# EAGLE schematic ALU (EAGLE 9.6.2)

## Sheet 1 of 8: Motherboard
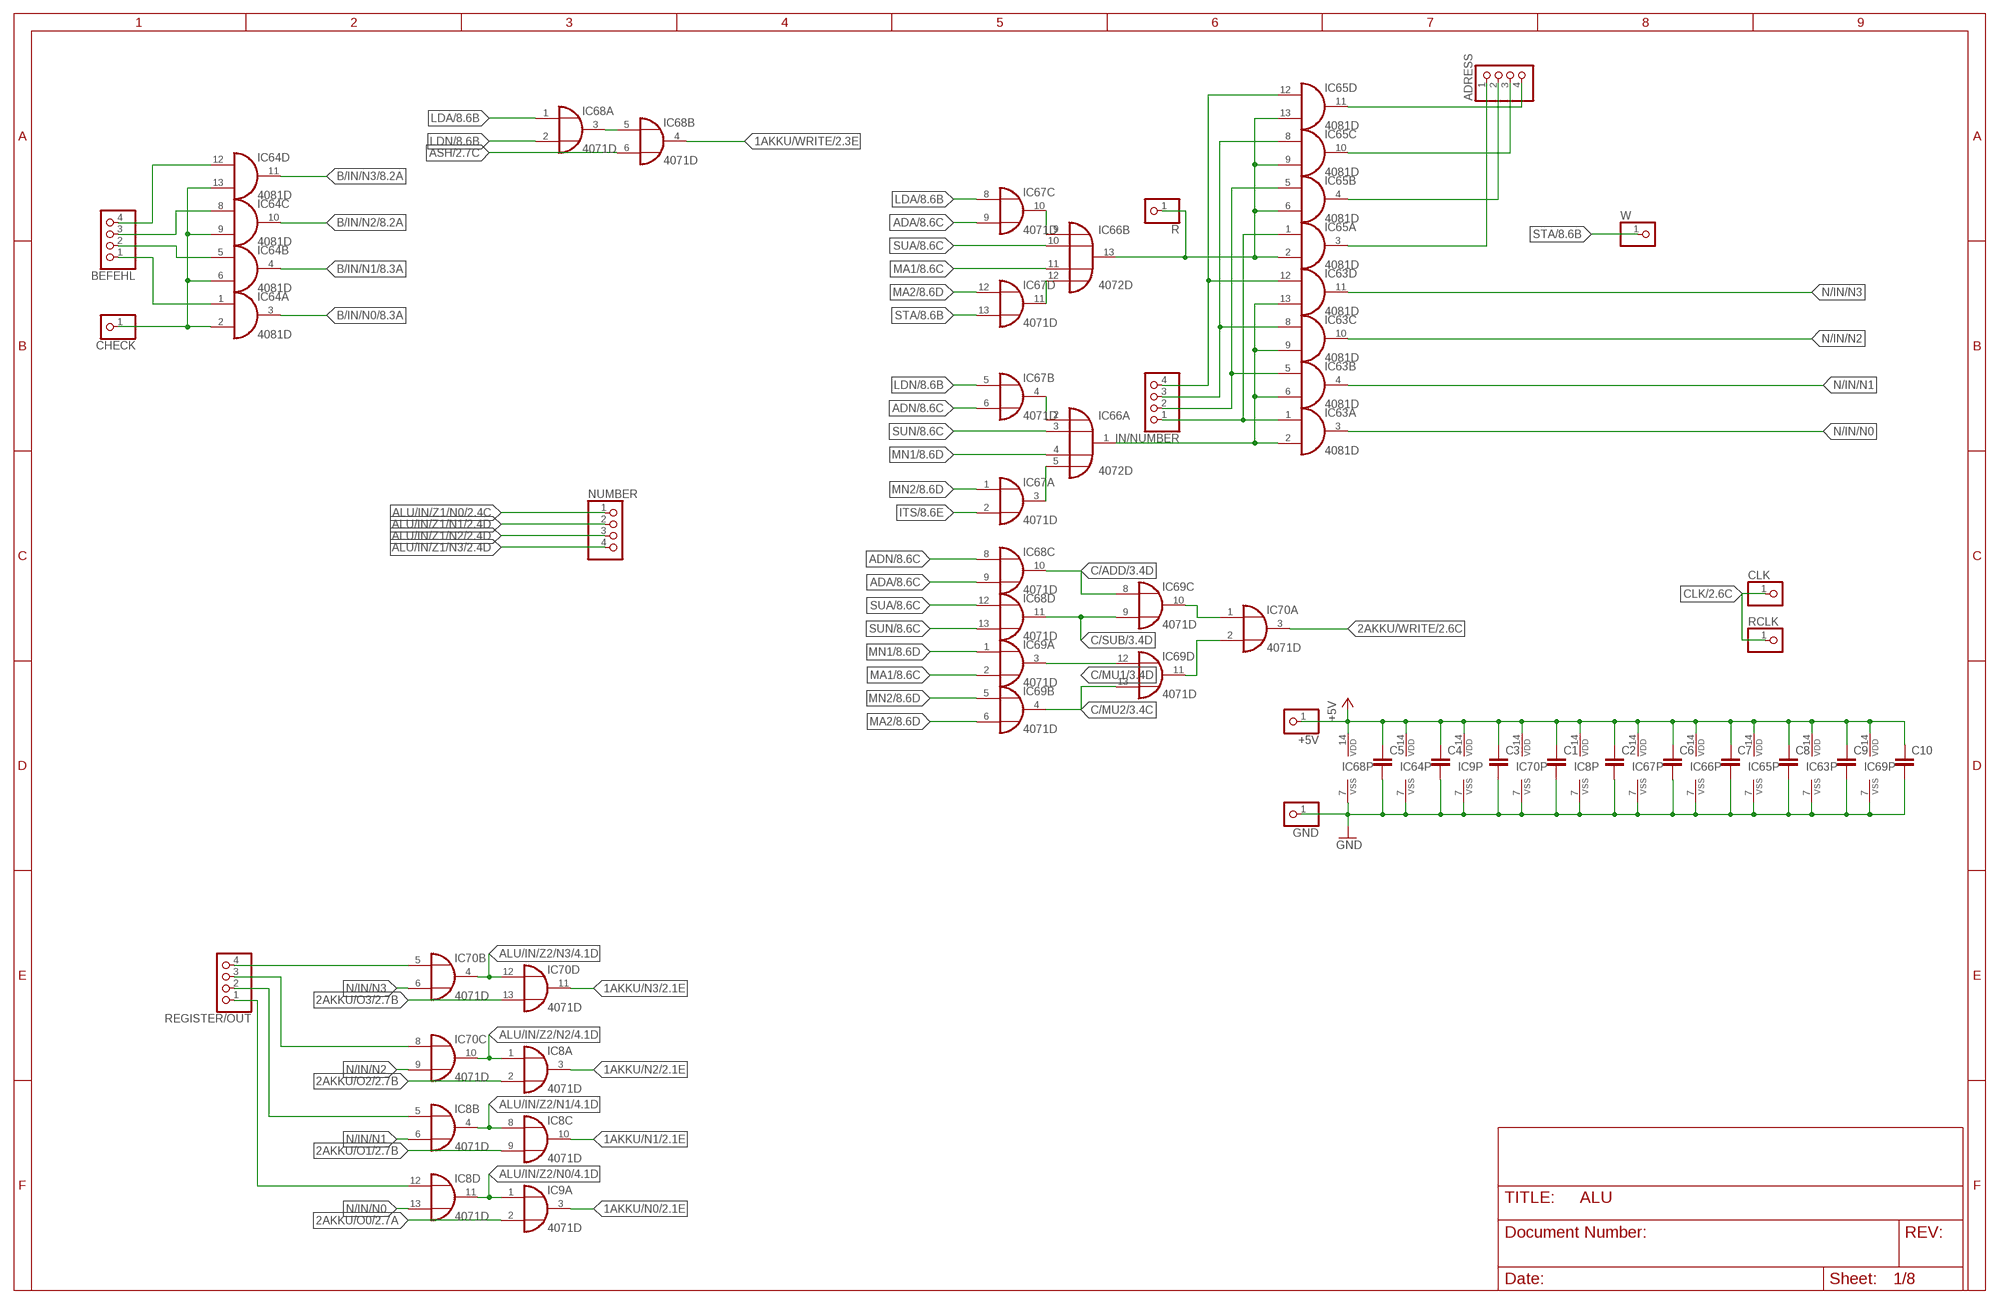
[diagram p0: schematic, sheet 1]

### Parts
+5V  PINHD-1X1  [1X01]
ADRESS  PINHD-1X4  [1X04]
BEFEHL  PINHD-1X4  [1X04]
C1  C-EUC0805  [C0805]
C2  C-EUC0805  [C0805]
C3  C-EUC0805  [C0805]
C4  C-EUC0805  [C0805]
C5  C-EUC0805  [C0805]
C6  C-EUC0805  [C0805]
C7  C-EUC0805  [C0805]
C8  C-EUC0805  [C0805]
C9  C-EUC0805  [C0805]
C10  C-EUC0805  [C0805]
CHECK  PINHD-1X1  [1X01]
CLK  PINHD-1X1  [1X01]
GND  PINHD-1X1  [1X01]
IC8  4071D  [SO14]
IC9  4071D  [SO14]
IC63  4081D  [SO14]
IC64  4081D  [SO14]
IC65  4081D  [SO14]
IC66  4072D  [SO14]
IC67  4071D  [SO14]
IC68  4071D  [SO14]
IC69  4071D  [SO14]
IC70  4071D  [SO14]
IN/NUMBER  PINHD-1X4  [1X04]
NUMBER  PINHD-1X4  [1X04]
R  PINHD-1X1  [1X01]
RCLK  PINHD-1X1  [1X01]
REGISTER/OUT  PINHD-1X4  [1X04]
W  PINHD-1X1  [1X01]

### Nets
1AKKU/N0: IC9.3(A:O) ; also sheet 2
1AKKU/N1: IC8.10(C:O) ; also sheet 2
1AKKU/N2: IC8.3(A:O) ; also sheet 2
1AKKU/N3: IC70.11(D:O) ; also sheet 2
1AKKU/WRITE: IC68.4(B:O) ; also sheet 2
2AKKU/O0: IC9.2(A:I1) ; also sheet 2
2AKKU/O1: IC8.9(C:I1) ; also sheet 2
2AKKU/O2: IC8.2(A:I1) ; also sheet 2
2AKKU/O3: IC70.13(D:I1) ; also sheet 2
2AKKU/WRITE: IC70.3(A:O) ; also sheet 2
+5V: +5V.1 C1.1 C2.1 C3.1 C4.1 C5.1 C6.1 C7.1 C8.1 C9.1 C10.1 IC8.14(P:VDD) IC9.14(P:VDD) IC63.14(P:VDD) IC64.14(P:VDD) IC65.14(P:VDD) IC66.14(P:VDD) IC67.14(P:VDD) IC68.14(P:VDD) IC69.14(P:VDD) IC70.14(P:VDD) ; also sheet 2,3,4,5,6,7,8
A/IN/N0: ADRESS.1 IC65.3(A:O)
A/IN/N1: ADRESS.2 IC65.4(B:O)
A/IN/N2: ADRESS.3 IC65.10(C:O)
A/IN/N3: ADRESS.4 IC65.11(D:O)
ADA: IC67.9(C:I1) IC68.9(C:I1) ; also sheet 8
ADN: IC67.6(B:I1) IC68.8(C:I0) ; also sheet 8
ALU/IN/Z1/N0: NUMBER.1 ; also sheet 2,4,5,6,7
ALU/IN/Z1/N1: NUMBER.2 ; also sheet 2,4,5,6,7
ALU/IN/Z1/N2: NUMBER.3 ; also sheet 2,4,5,6,7
ALU/IN/Z1/N3: NUMBER.4 ; also sheet 2,4,5,6,7
ALU/IN/Z2/N0: IC8.11(D:O) IC9.1(A:I0) ; also sheet 4,5,6,7
ALU/IN/Z2/N1: IC8.4(B:O) IC8.8(C:I0) ; also sheet 4,5,6,7
ALU/IN/Z2/N2: IC8.1(A:I0) IC70.10(C:O) ; also sheet 4,5,6,7
ALU/IN/Z2/N3: IC70.4(B:O) IC70.12(D:I0) ; also sheet 4,5,6,7
ASH: IC68.6(B:I1) ; also sheet 2,8
B/IN/N0: IC64.3(A:O) ; also sheet 8
B/IN/N1: IC64.4(B:O) ; also sheet 8
B/IN/N2: IC64.10(C:O) ; also sheet 8
B/IN/N3: IC64.11(D:O) ; also sheet 8
C/ADD: IC68.10(C:O) IC69.8(C:I0) ; also sheet 3
C/MU1: IC69.3(A:O) IC69.12(D:I0) ; also sheet 3
C/MU2: IC69.4(B:O) IC69.13(D:I1) ; also sheet 3
C/SUB: IC68.11(D:O) IC69.9(C:I1) ; also sheet 3
CLK: CLK.1 RCLK.1 ; also sheet 2,3
GND: C1.2 C2.2 C3.2 C4.2 C5.2 C6.2 C7.2 C8.2 C9.2 C10.2 GND.1 IC8.7(P:VSS) IC9.7(P:VSS) IC63.7(P:VSS) IC64.7(P:VSS) IC65.7(P:VSS) IC66.7(P:VSS) IC67.7(P:VSS) IC68.7(P:VSS) IC69.7(P:VSS) IC70.7(P:VSS) ; also sheet 2,3,4,5,6,7,8
ITS: IC67.2(A:I1) ; also sheet 8
LDA: IC67.8(C:I0) IC68.1(A:I0) ; also sheet 8
LDN: IC67.5(B:I0) IC68.2(A:I1) ; also sheet 8
MA1: IC66.11(B:I2) IC69.2(A:I1) ; also sheet 8
MA2: IC67.12(D:I0) IC69.6(B:I1) ; also sheet 8
MN1: IC66.4(A:I2) IC69.1(A:I0) ; also sheet 8
MN2: IC67.1(A:I0) IC69.5(B:I0) ; also sheet 8
N$14: IC70.5(B:I0) REGISTER/OUT.4
N$19: IC70.8(C:I0) REGISTER/OUT.3
N$20: IC8.5(B:I0) REGISTER/OUT.2
N$22: IC8.12(D:I0) REGISTER/OUT.1
N$141: BEFEHL.4 IC64.12(D:I0)
N$143: BEFEHL.3 IC64.8(C:I0)
N$145: BEFEHL.2 IC64.5(B:I0)
N$147: BEFEHL.1 IC64.1(A:I0)
N$149: CHECK.1 IC64.2(A:I1) IC64.6(B:I1) IC64.9(C:I1) IC64.13(D:I1)
N$150: IC63.12(D:I0) IC65.12(D:I0) IN/NUMBER.4
N$151: IC63.8(C:I0) IC65.8(C:I0) IN/NUMBER.3
N$152: IC63.5(B:I0) IC65.5(B:I0) IN/NUMBER.2
N$153: IC63.1(A:I0) IC65.1(A:I0) IN/NUMBER.1
N$154: IC63.2(A:I1) IC63.6(B:I1) IC63.9(C:I1) IC63.13(D:I1) IC66.1(A:O)
N$155: IC68.3(A:O) IC68.5(B:I0)
N$156: IC66.5(A:I3) IC67.3(A:O)
N$158: IC66.2(A:I0) IC67.4(B:O)
N$159: IC65.2(A:I1) IC65.6(B:I1) IC65.9(C:I1) IC65.13(D:I1) IC66.13(B:O) R.1
N$160: IC66.9(B:I0) IC67.10(C:O)
N$161: IC66.12(B:I3) IC67.11(D:O)
N$173: IC69.10(C:O) IC70.1(A:I0)
N$174: IC69.11(D:O) IC70.2(A:I1)
N/IN/N0: IC8.13(D:I1) IC63.3(A:O)
N/IN/N1: IC8.6(B:I1) IC63.4(B:O)
N/IN/N2: IC63.10(C:O) IC70.9(C:I1)
N/IN/N3: IC63.11(D:O) IC70.6(B:I1)
STA: IC67.13(D:I1) W.1 ; also sheet 8
SUA: IC66.10(B:I1) IC68.12(D:I0) ; also sheet 8
SUN: IC66.3(A:I1) IC68.13(D:I1) ; also sheet 8

## Sheet 2 of 8: Akkumulator
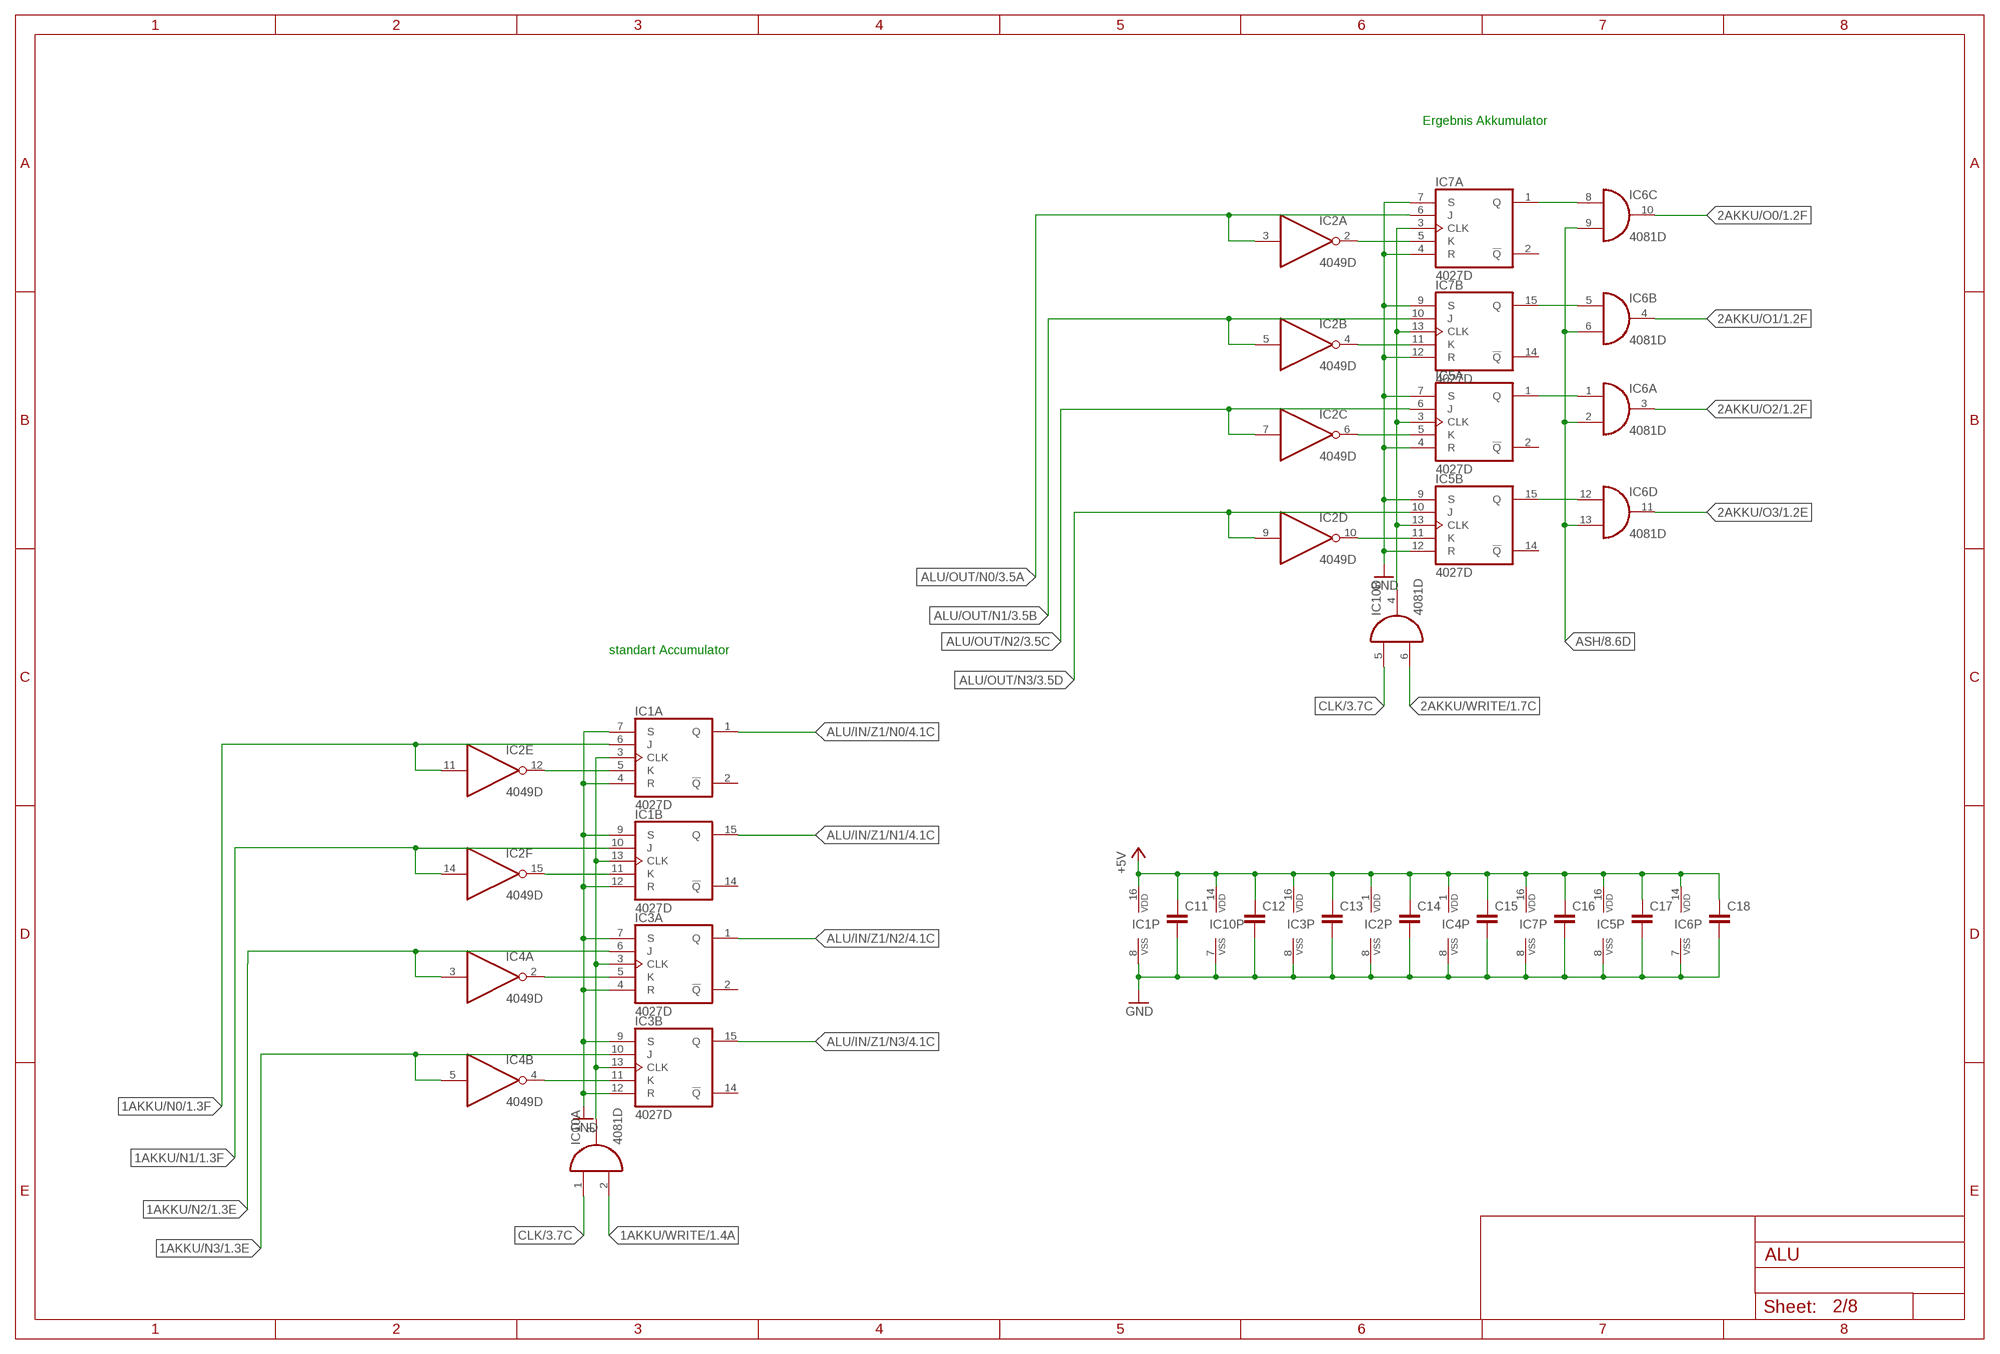
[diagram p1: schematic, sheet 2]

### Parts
C11  C-EUC0805  [C0805]
C12  C-EUC0805  [C0805]
C13  C-EUC0805  [C0805]
C14  C-EUC0805  [C0805]
C15  C-EUC0805  [C0805]
C16  C-EUC0805  [C0805]
C17  C-EUC0805  [C0805]
C18  C-EUC0805  [C0805]
IC1  4027D  [SO16]
IC2  4049D  [SO16]
IC3  4027D  [SO16]
IC4  4049D  [SO16]
IC5  4027D  [SO16]
IC6  4081D  [SO14]
IC7  4027D  [SO16]
IC10  4081D  [SO14]

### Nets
1AKKU/N0: IC1.6(A:J) IC2.11(E:I) ; also sheet 1
1AKKU/N1: IC1.10(B:J) IC2.14(F:I) ; also sheet 1
1AKKU/N2: IC3.6(A:J) IC4.3(A:I) ; also sheet 1
1AKKU/N3: IC3.10(B:J) IC4.5(B:I) ; also sheet 1
1AKKU/WRITE: IC10.2(A:I1) ; also sheet 1
2AKKU/O0: IC6.10(C:O) ; also sheet 1
2AKKU/O1: IC6.4(B:O) ; also sheet 1
2AKKU/O2: IC6.3(A:O) ; also sheet 1
2AKKU/O3: IC6.11(D:O) ; also sheet 1
2AKKU/WRITE: IC10.6(B:I1) ; also sheet 1
+5V: C11.1 C12.1 C13.1 C14.1 C15.1 C16.1 C17.1 C18.1 IC1.16(P:VDD) IC2.1(P:VDD) IC3.16(P:VDD) IC4.1(P:VDD) IC5.16(P:VDD) IC6.14(P:VDD) IC7.16(P:VDD) IC10.14(P:VDD) ; also sheet 1,3,4,5,6,7,8
ALU/IN/Z1/N0: IC1.1(A:Q) ; also sheet 1,4,5,6,7
ALU/IN/Z1/N1: IC1.15(B:Q) ; also sheet 1,4,5,6,7
ALU/IN/Z1/N2: IC3.1(A:Q) ; also sheet 1,4,5,6,7
ALU/IN/Z1/N3: IC3.15(B:Q) ; also sheet 1,4,5,6,7
ALU/OUT/N0: IC2.3(A:I) IC7.6(A:J) ; also sheet 3
ALU/OUT/N1: IC2.5(B:I) IC7.10(B:J) ; also sheet 3
ALU/OUT/N2: IC2.7(C:I) IC5.6(A:J) ; also sheet 3
ALU/OUT/N3: IC2.9(D:I) IC5.10(B:J) ; also sheet 3
ASH: IC6.2(A:I1) IC6.6(B:I1) IC6.9(C:I1) IC6.13(D:I1) ; also sheet 1,8
CLK: IC10.1(A:I0) IC10.5(B:I0) ; also sheet 1,3
GND: C11.2 C12.2 C13.2 C14.2 C15.2 C16.2 C17.2 C18.2 IC1.4(A:R) IC1.7(A:S) IC1.8(P:VSS) IC1.9(B:S) IC1.12(B:R) IC2.8(P:VSS) IC3.4(A:R) IC3.7(A:S) IC3.8(P:VSS) IC3.9(B:S) IC3.12(B:R) IC4.8(P:VSS) IC5.4(A:R) IC5.7(A:S) IC5.8(P:VSS) IC5.9(B:S) IC5.12(B:R) IC6.7(P:VSS) IC7.4(A:R) IC7.7(A:S) IC7.8(P:VSS) IC7.9(B:S) IC7.12(B:R) IC10.7(P:VSS) ; also sheet 1,3,4,5,6,7,8
N$1: IC1.5(A:K) IC2.12(E:O)
N$2: IC5.3(A:CLK) IC5.13(B:CLK) IC7.3(A:CLK) IC7.13(B:CLK) IC10.4(B:O)
N$3: IC1.3(A:CLK) IC1.13(B:CLK) IC3.3(A:CLK) IC3.13(B:CLK) IC10.3(A:O)
N$4: IC1.11(B:K) IC2.15(F:O)
N$5: IC3.5(A:K) IC4.2(A:O)
N$6: IC6.8(C:I0) IC7.1(A:Q)
N$7: IC6.5(B:I0) IC7.15(B:Q)
N$8: IC3.11(B:K) IC4.4(B:O)
N$9: IC2.6(C:O) IC5.5(A:K)
N$10: IC5.1(A:Q) IC6.1(A:I0)
N$11: IC5.15(B:Q) IC6.12(D:I0)
N$12: IC2.10(D:O) IC5.11(B:K)
N$13: IC2.2(A:O) IC7.5(A:K)
N$16: IC2.4(B:O) IC7.11(B:K)
Unconnected: IC1.2(A:!Q) IC1.14(B:!Q) IC3.2(A:!Q) IC3.14(B:!Q) IC5.2(A:!Q) IC5.14(B:!Q) IC7.2(A:!Q) IC7.14(B:!Q)

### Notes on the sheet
- Ergebnis Akkumulator
- standart Accumulator

## Sheet 3 of 8: ALU
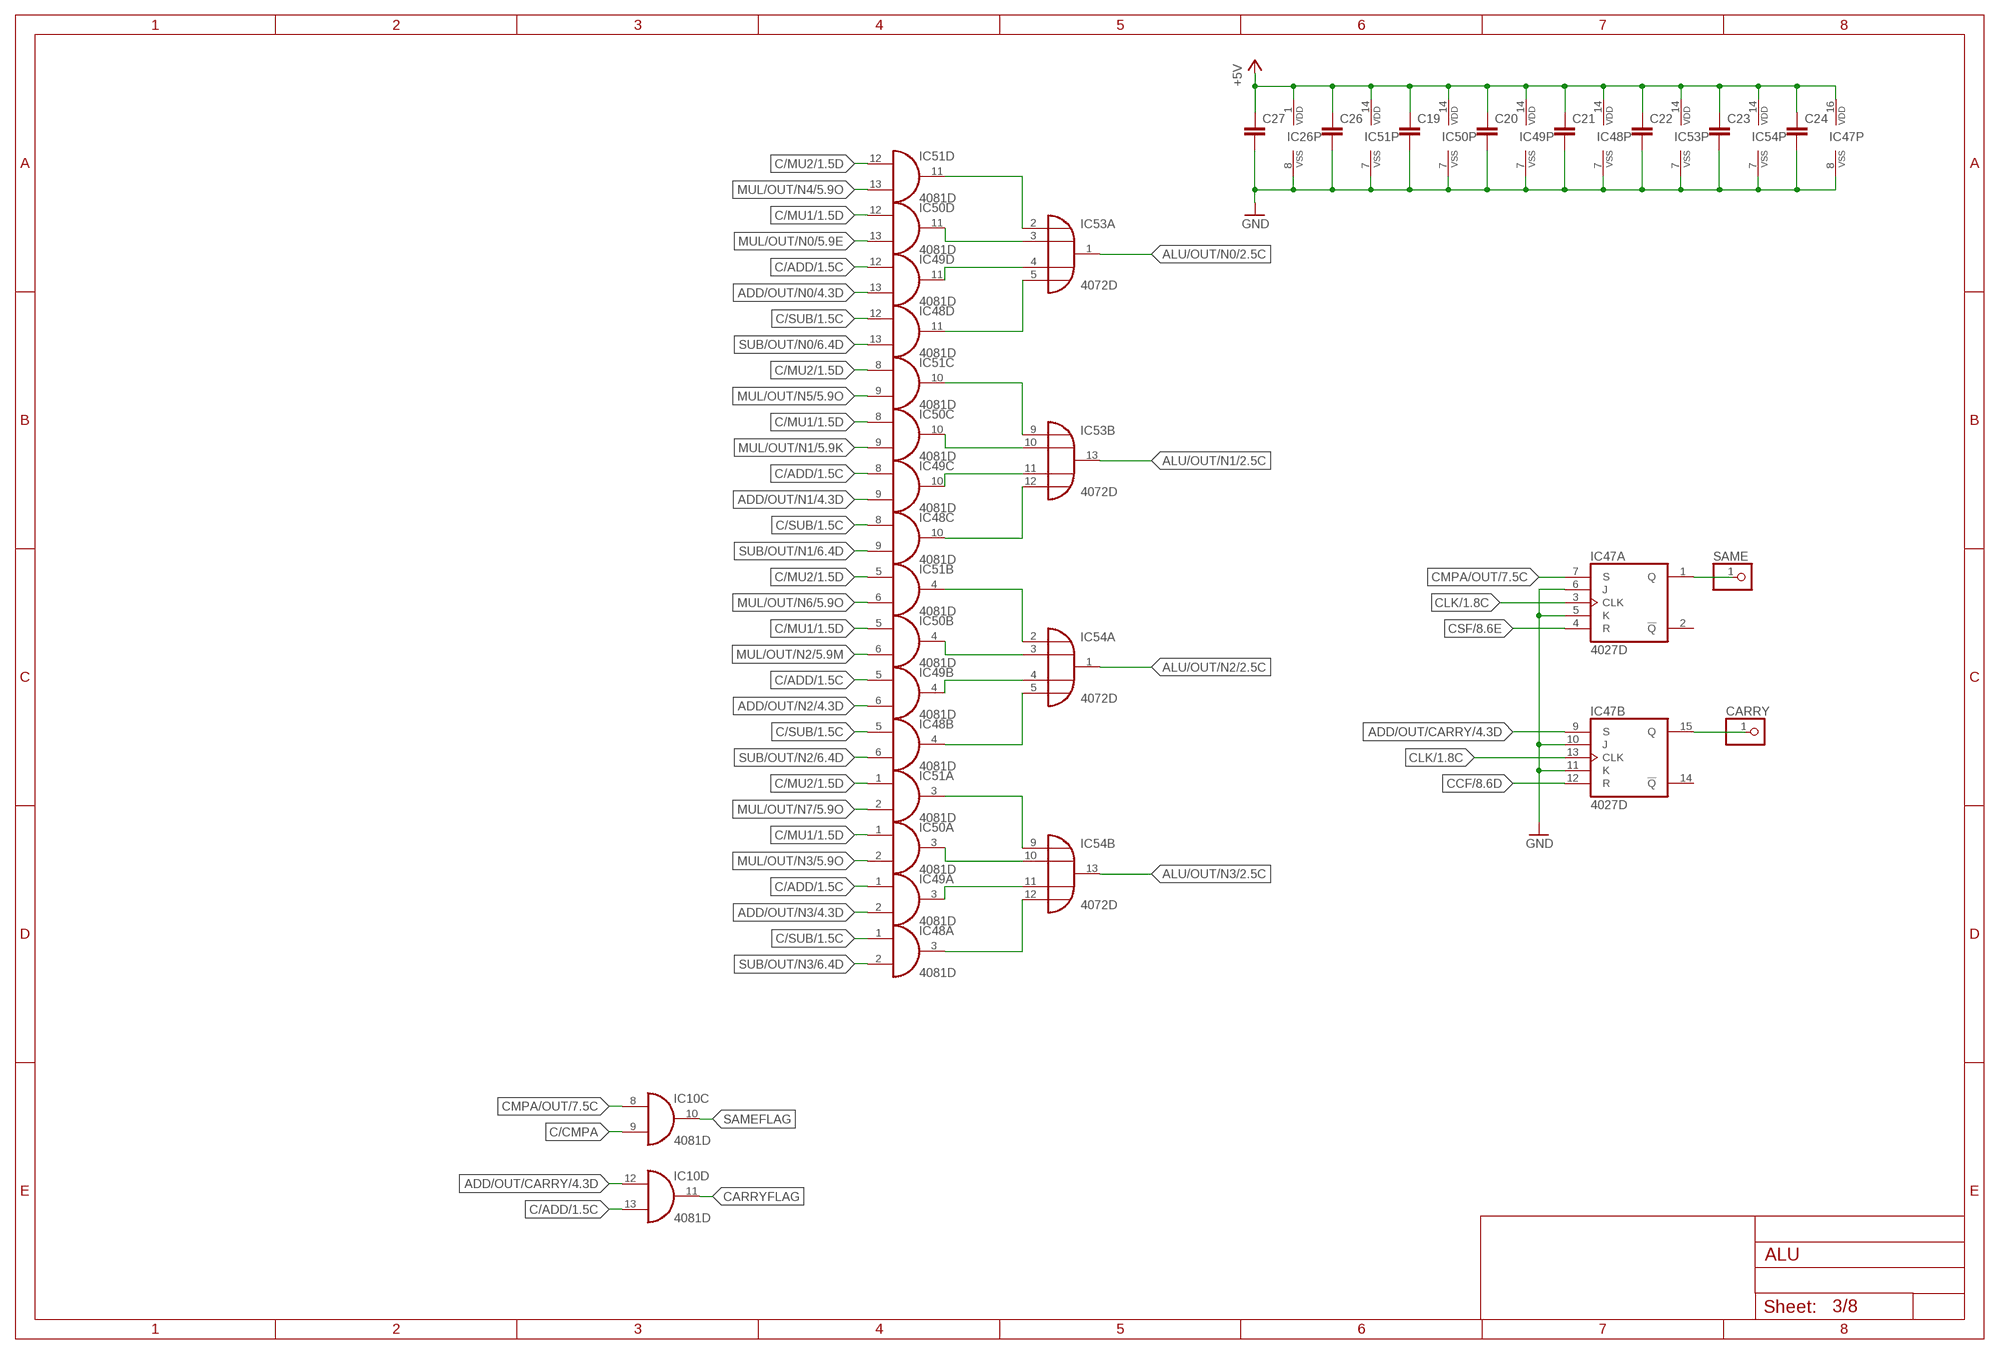
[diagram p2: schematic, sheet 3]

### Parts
C19  C-EUC0805  [C0805]
C20  C-EUC0805  [C0805]
C21  C-EUC0805  [C0805]
C22  C-EUC0805  [C0805]
C23  C-EUC0805  [C0805]
C24  C-EUC0805  [C0805]
C26  C-EUC0805  [C0805]
C27  C-EUC0805  [C0805]
CARRY  PINHD-1X1  [1X01]
IC26  4049D  [SO16]
IC47  4027D  [SO16]
IC48  4081D  [SO14]
IC49  4081D  [SO14]
IC50  4081D  [SO14]
IC51  4081D  [SO14]
IC53  4072D  [SO14]
IC54  4072D  [SO14]
SAME  PINHD-1X1  [1X01]

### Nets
+5V: C19.1 C20.1 C21.1 C22.1 C23.1 C24.1 C26.1 C27.1 IC26.1(P:VDD) IC47.16(P:VDD) IC48.14(P:VDD) IC49.14(P:VDD) IC50.14(P:VDD) IC51.14(P:VDD) IC53.14(P:VDD) IC54.14(P:VDD) ; also sheet 1,2,4,5,6,7,8
ADD/OUT/CARRY: IC10.12(D:I0) IC47.9(B:S) ; also sheet 4
ADD/OUT/N0: IC49.13(D:I1) ; also sheet 4
ADD/OUT/N1: IC49.9(C:I1) ; also sheet 4
ADD/OUT/N2: IC49.6(B:I1) ; also sheet 4
ADD/OUT/N3: IC49.2(A:I1) ; also sheet 4
ALU/OUT/N0: IC53.1(A:O) ; also sheet 2
ALU/OUT/N1: IC53.13(B:O) ; also sheet 2
ALU/OUT/N2: IC54.1(A:O) ; also sheet 2
ALU/OUT/N3: IC54.13(B:O) ; also sheet 2
C/ADD: IC10.13(D:I1) IC49.1(A:I0) IC49.5(B:I0) IC49.8(C:I0) IC49.12(D:I0) ; also sheet 1
C/CMPA: IC10.9(C:I1)
C/MU1: IC50.1(A:I0) IC50.5(B:I0) IC50.8(C:I0) IC50.12(D:I0) ; also sheet 1
C/MU2: IC51.1(A:I0) IC51.5(B:I0) IC51.8(C:I0) IC51.12(D:I0) ; also sheet 1
C/SUB: IC48.1(A:I0) IC48.5(B:I0) IC48.8(C:I0) IC48.12(D:I0) ; also sheet 1
CARRYFLAG: IC10.11(D:O)
CCF: IC47.12(B:R) ; also sheet 8
CLK: IC47.3(A:CLK) IC47.13(B:CLK) ; also sheet 1,2
CMPA/OUT: IC10.8(C:I0) IC47.7(A:S) ; also sheet 7
CSF: IC47.4(A:R) ; also sheet 8
GND: C19.2 C20.2 C21.2 C22.2 C23.2 C24.2 C26.2 C27.2 IC26.8(P:VSS) IC47.5(A:K) IC47.6(A:J) IC47.8(P:VSS) IC47.10(B:J) IC47.11(B:K) IC48.7(P:VSS) IC49.7(P:VSS) IC50.7(P:VSS) IC51.7(P:VSS) IC53.7(P:VSS) IC54.7(P:VSS) ; also sheet 1,2,4,5,6,7,8
MUL/OUT/N0: IC50.13(D:I1) ; also sheet 5
MUL/OUT/N1: IC50.9(C:I1) ; also sheet 5
MUL/OUT/N2: IC50.6(B:I1) ; also sheet 5
MUL/OUT/N3: IC50.2(A:I1) ; also sheet 5
MUL/OUT/N4: IC51.13(D:I1) ; also sheet 5
MUL/OUT/N5: IC51.9(C:I1) ; also sheet 5
MUL/OUT/N6: IC51.6(B:I1) ; also sheet 5
MUL/OUT/N7: IC51.2(A:I1) ; also sheet 5
N$106: IC49.11(D:O) IC53.4(A:I2)
N$120: IC50.11(D:O) IC53.3(A:I1)
N$121: IC51.11(D:O) IC53.2(A:I0)
N$122: IC48.11(D:O) IC53.5(A:I3)
N$123: IC49.10(C:O) IC53.11(B:I2)
N$124: IC50.10(C:O) IC53.10(B:I1)
N$125: IC51.10(C:O) IC53.9(B:I0)
N$126: IC48.10(C:O) IC53.12(B:I3)
N$133: IC50.4(B:O) IC54.3(A:I1)
N$134: IC49.4(B:O) IC54.4(A:I2)
N$135: IC48.4(B:O) IC54.5(A:I3)
N$136: IC51.4(B:O) IC54.2(A:I0)
N$137: IC50.3(A:O) IC54.10(B:I1)
N$138: IC49.3(A:O) IC54.11(B:I2)
N$139: IC51.3(A:O) IC54.9(B:I0)
N$140: IC48.3(A:O) IC54.12(B:I3)
N$167: IC47.1(A:Q) SAME.1
N$171: CARRY.1 IC47.15(B:Q)
SAMEFLAG: IC10.10(C:O)
SUB/OUT/N0: IC48.13(D:I1) ; also sheet 6
SUB/OUT/N1: IC48.9(C:I1) ; also sheet 6
SUB/OUT/N2: IC48.6(B:I1) ; also sheet 6
SUB/OUT/N3: IC48.2(A:I1) ; also sheet 6
Unconnected: IC47.2(A:!Q) IC47.14(B:!Q)

## Sheet 4 of 8: Addirer
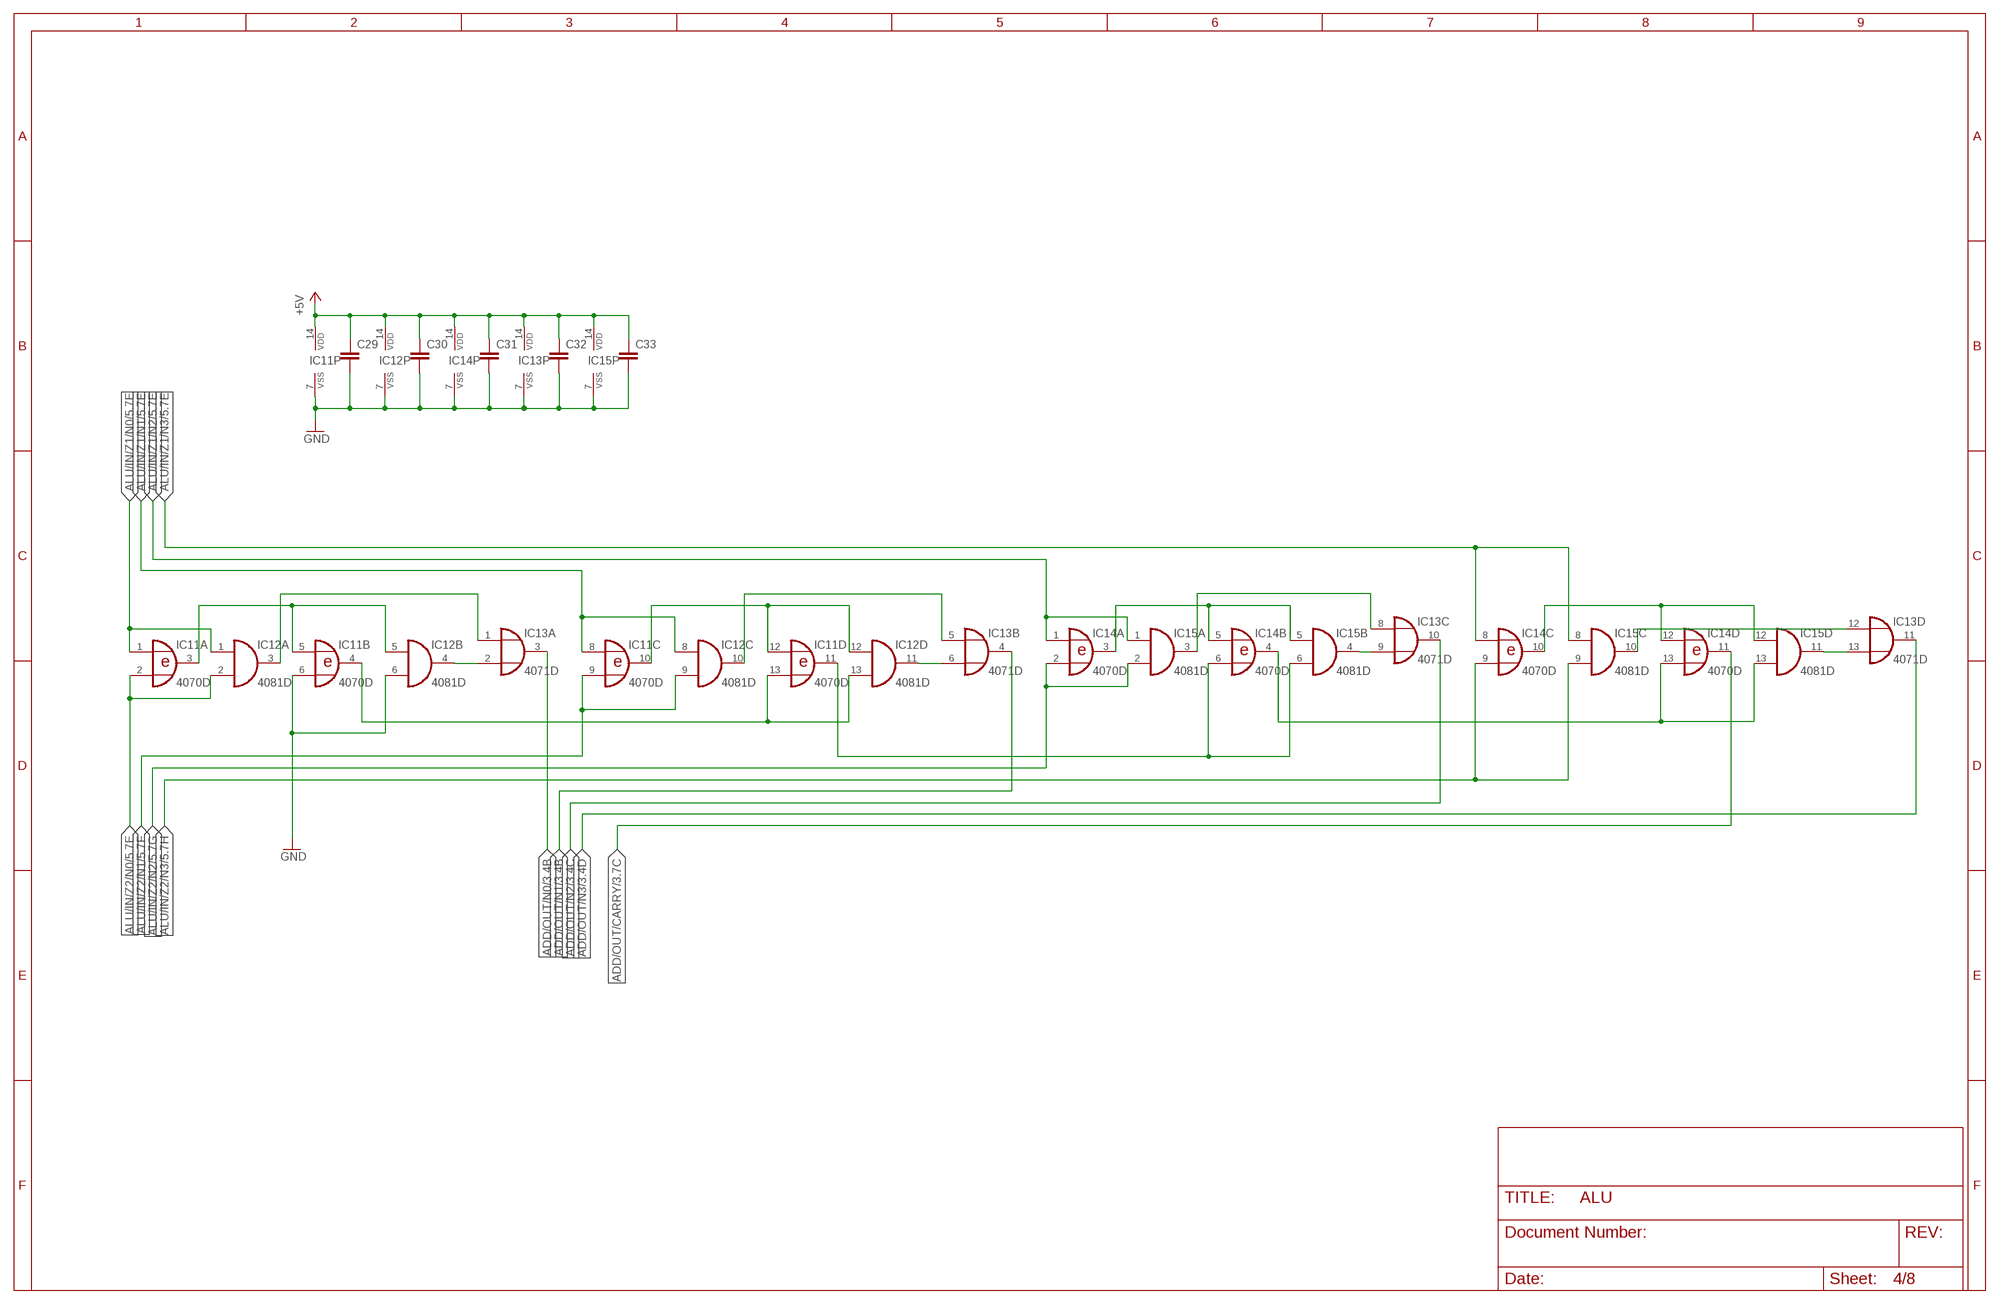
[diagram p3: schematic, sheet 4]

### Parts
C29  C-EUC0805  [C0805]
C30  C-EUC0805  [C0805]
C31  C-EUC0805  [C0805]
C32  C-EUC0805  [C0805]
C33  C-EUC0805  [C0805]
IC11  4070D  [SO14]
IC12  4081D  [SO14]
IC13  4071D  [SO14]
IC14  4070D  [SO14]
IC15  4081D  [SO14]

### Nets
+5V: C29.1 C30.1 C31.1 C32.1 C33.1 IC11.14(P:VDD) IC12.14(P:VDD) IC13.14(P:VDD) IC14.14(P:VDD) IC15.14(P:VDD) ; also sheet 1,2,3,5,6,7,8
ADD/OUT/CARRY: IC14.11(D:O) ; also sheet 3
ADD/OUT/N0: IC13.3(A:O) ; also sheet 3
ADD/OUT/N1: IC13.4(B:O) ; also sheet 3
ADD/OUT/N2: IC13.10(C:O) ; also sheet 3
ADD/OUT/N3: IC13.11(D:O) ; also sheet 3
ALU/IN/Z1/N0: IC11.1(A:I0) IC12.1(A:I0) ; also sheet 1,2,5,6,7
ALU/IN/Z1/N1: IC11.8(C:I0) IC12.8(C:I0) ; also sheet 1,2,5,6,7
ALU/IN/Z1/N2: IC14.1(A:I0) IC15.1(A:I0) ; also sheet 1,2,5,6,7
ALU/IN/Z1/N3: IC14.8(C:I0) IC15.8(C:I0) ; also sheet 1,2,5,6,7
ALU/IN/Z2/N0: IC11.2(A:I1) IC12.2(A:I1) ; also sheet 1,5,6,7
ALU/IN/Z2/N1: IC11.9(C:I1) IC12.9(C:I1) ; also sheet 1,5,6,7
ALU/IN/Z2/N2: IC14.2(A:I1) IC15.2(A:I1) ; also sheet 1,5,6,7
ALU/IN/Z2/N3: IC14.9(C:I1) IC15.9(C:I1) ; also sheet 1,5,6,7
GND: C29.2 C30.2 C31.2 C32.2 C33.2 IC11.6(B:I1) IC11.7(P:VSS) IC12.6(B:I1) IC12.7(P:VSS) IC13.7(P:VSS) IC14.7(P:VSS) IC15.7(P:VSS) ; also sheet 1,2,3,5,6,7,8
N$21: IC11.3(A:O) IC11.5(B:I0) IC12.5(B:I0)
N$25: IC12.3(A:O) IC13.1(A:I0)
N$29: IC12.4(B:O) IC13.2(A:I1)
N$31: IC11.4(B:O) IC11.13(D:I1) IC12.13(D:I1)
N$39: IC11.11(D:O) IC14.6(B:I1) IC15.6(B:I1)
N$40: IC11.10(C:O) IC11.12(D:I0) IC12.12(D:I0)
N$41: IC12.10(C:O) IC13.5(B:I0)
N$42: IC12.11(D:O) IC13.6(B:I1)
N$48: IC14.3(A:O) IC14.5(B:I0) IC15.5(B:I0)
N$49: IC14.4(B:O) IC14.13(D:I1) IC15.13(D:I1)
N$50: IC13.9(C:I1) IC15.4(B:O)
N$51: IC13.8(C:I0) IC15.3(A:O)
N$54: IC14.10(C:O) IC14.12(D:I0) IC15.12(D:I0)
N$55: IC13.12(D:I0) IC15.10(C:O)
N$56: IC13.13(D:I1) IC15.11(D:O)

## Sheet 5 of 8: multiplier
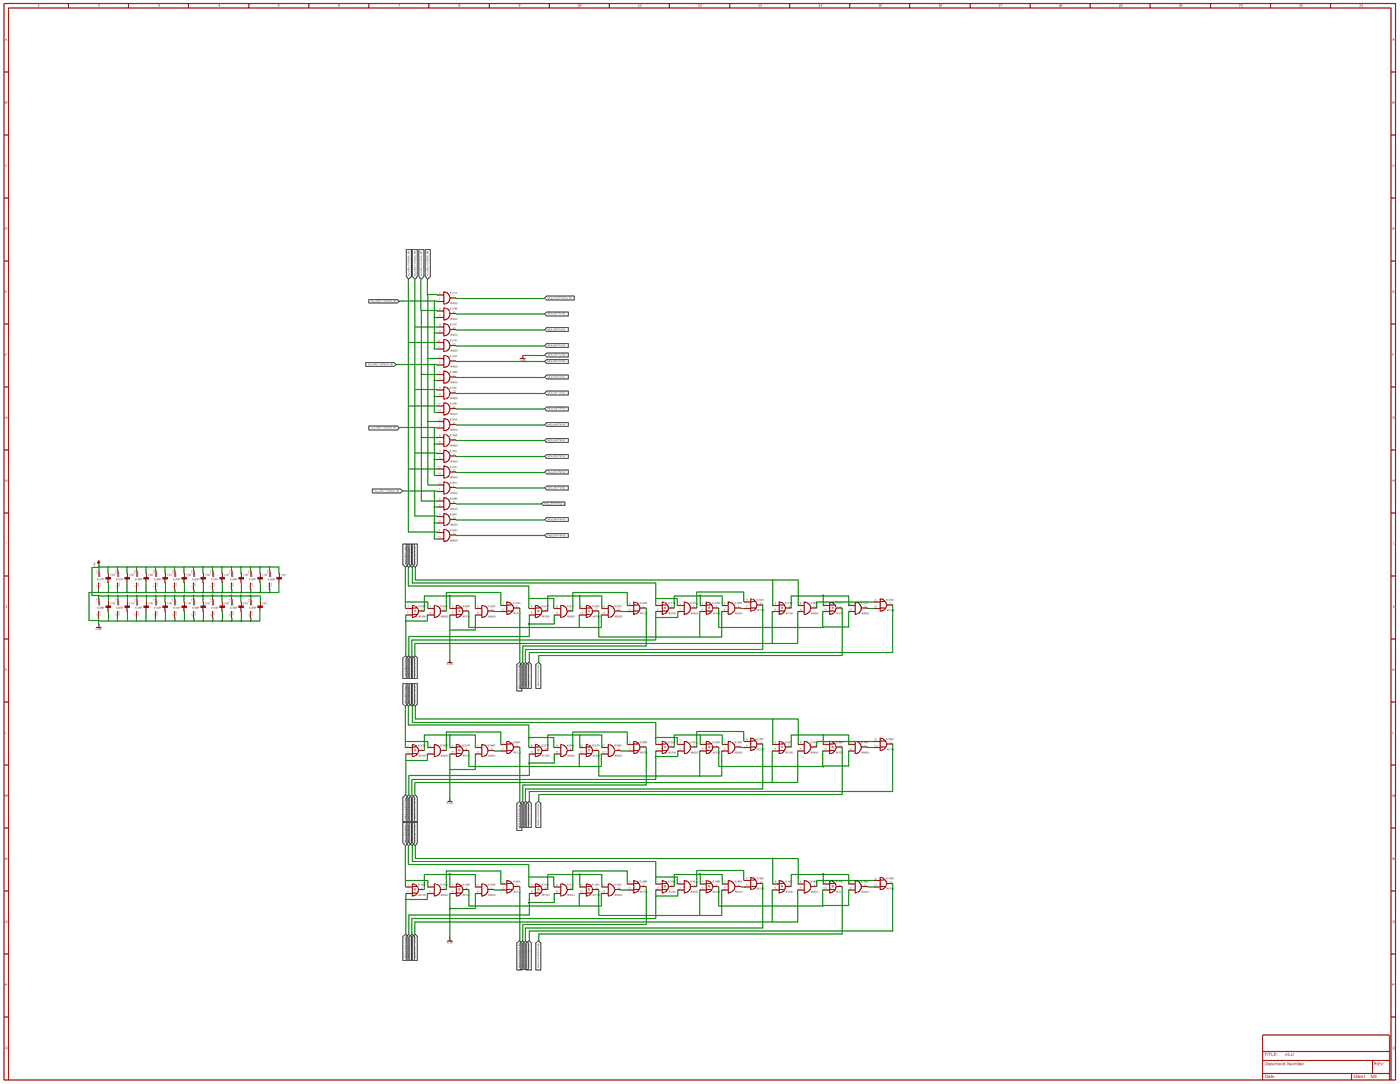
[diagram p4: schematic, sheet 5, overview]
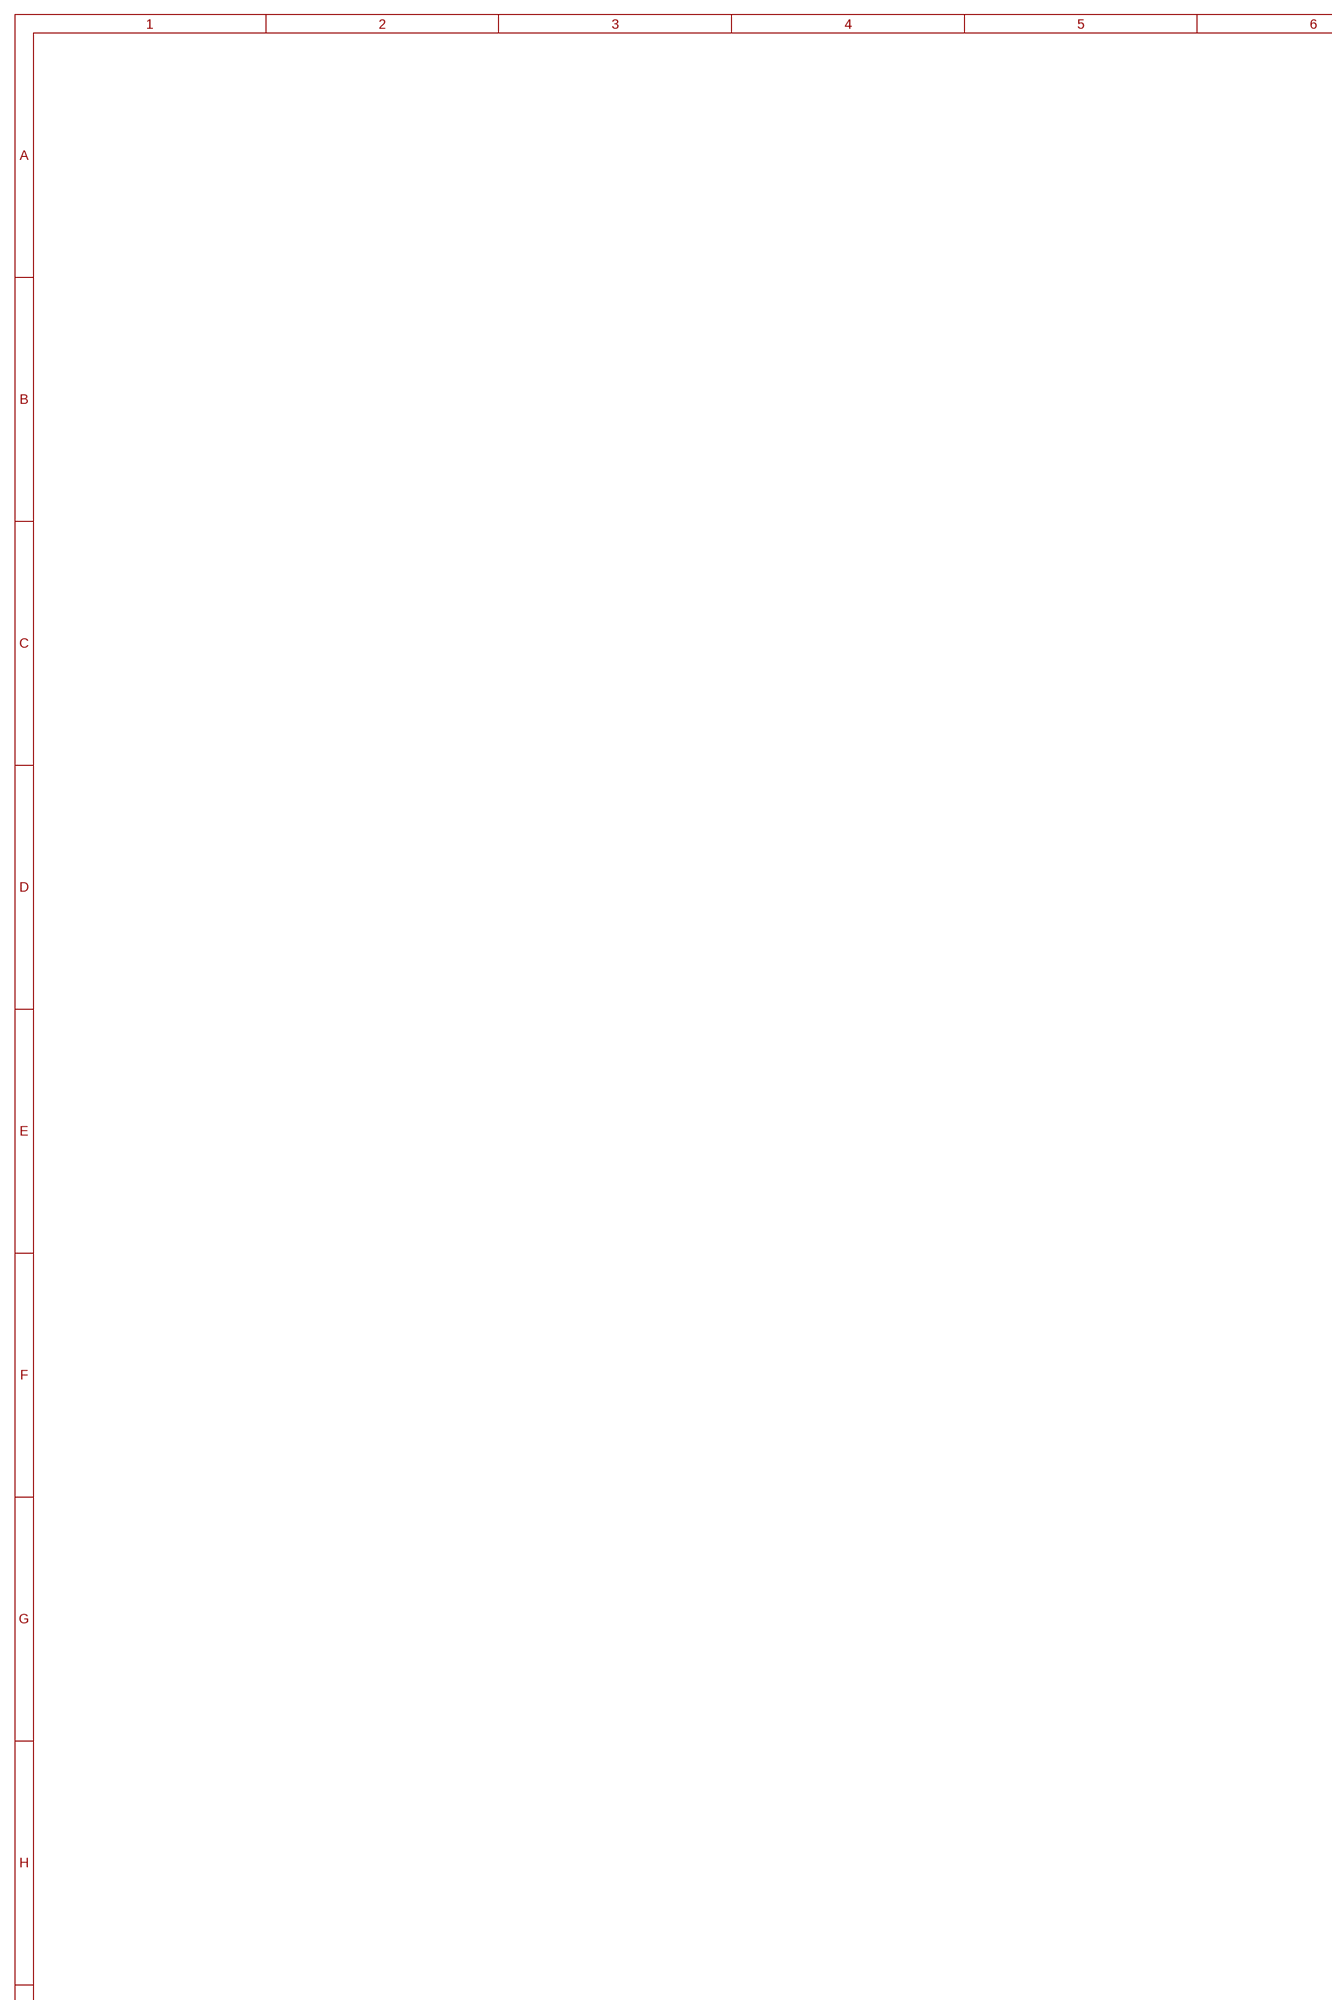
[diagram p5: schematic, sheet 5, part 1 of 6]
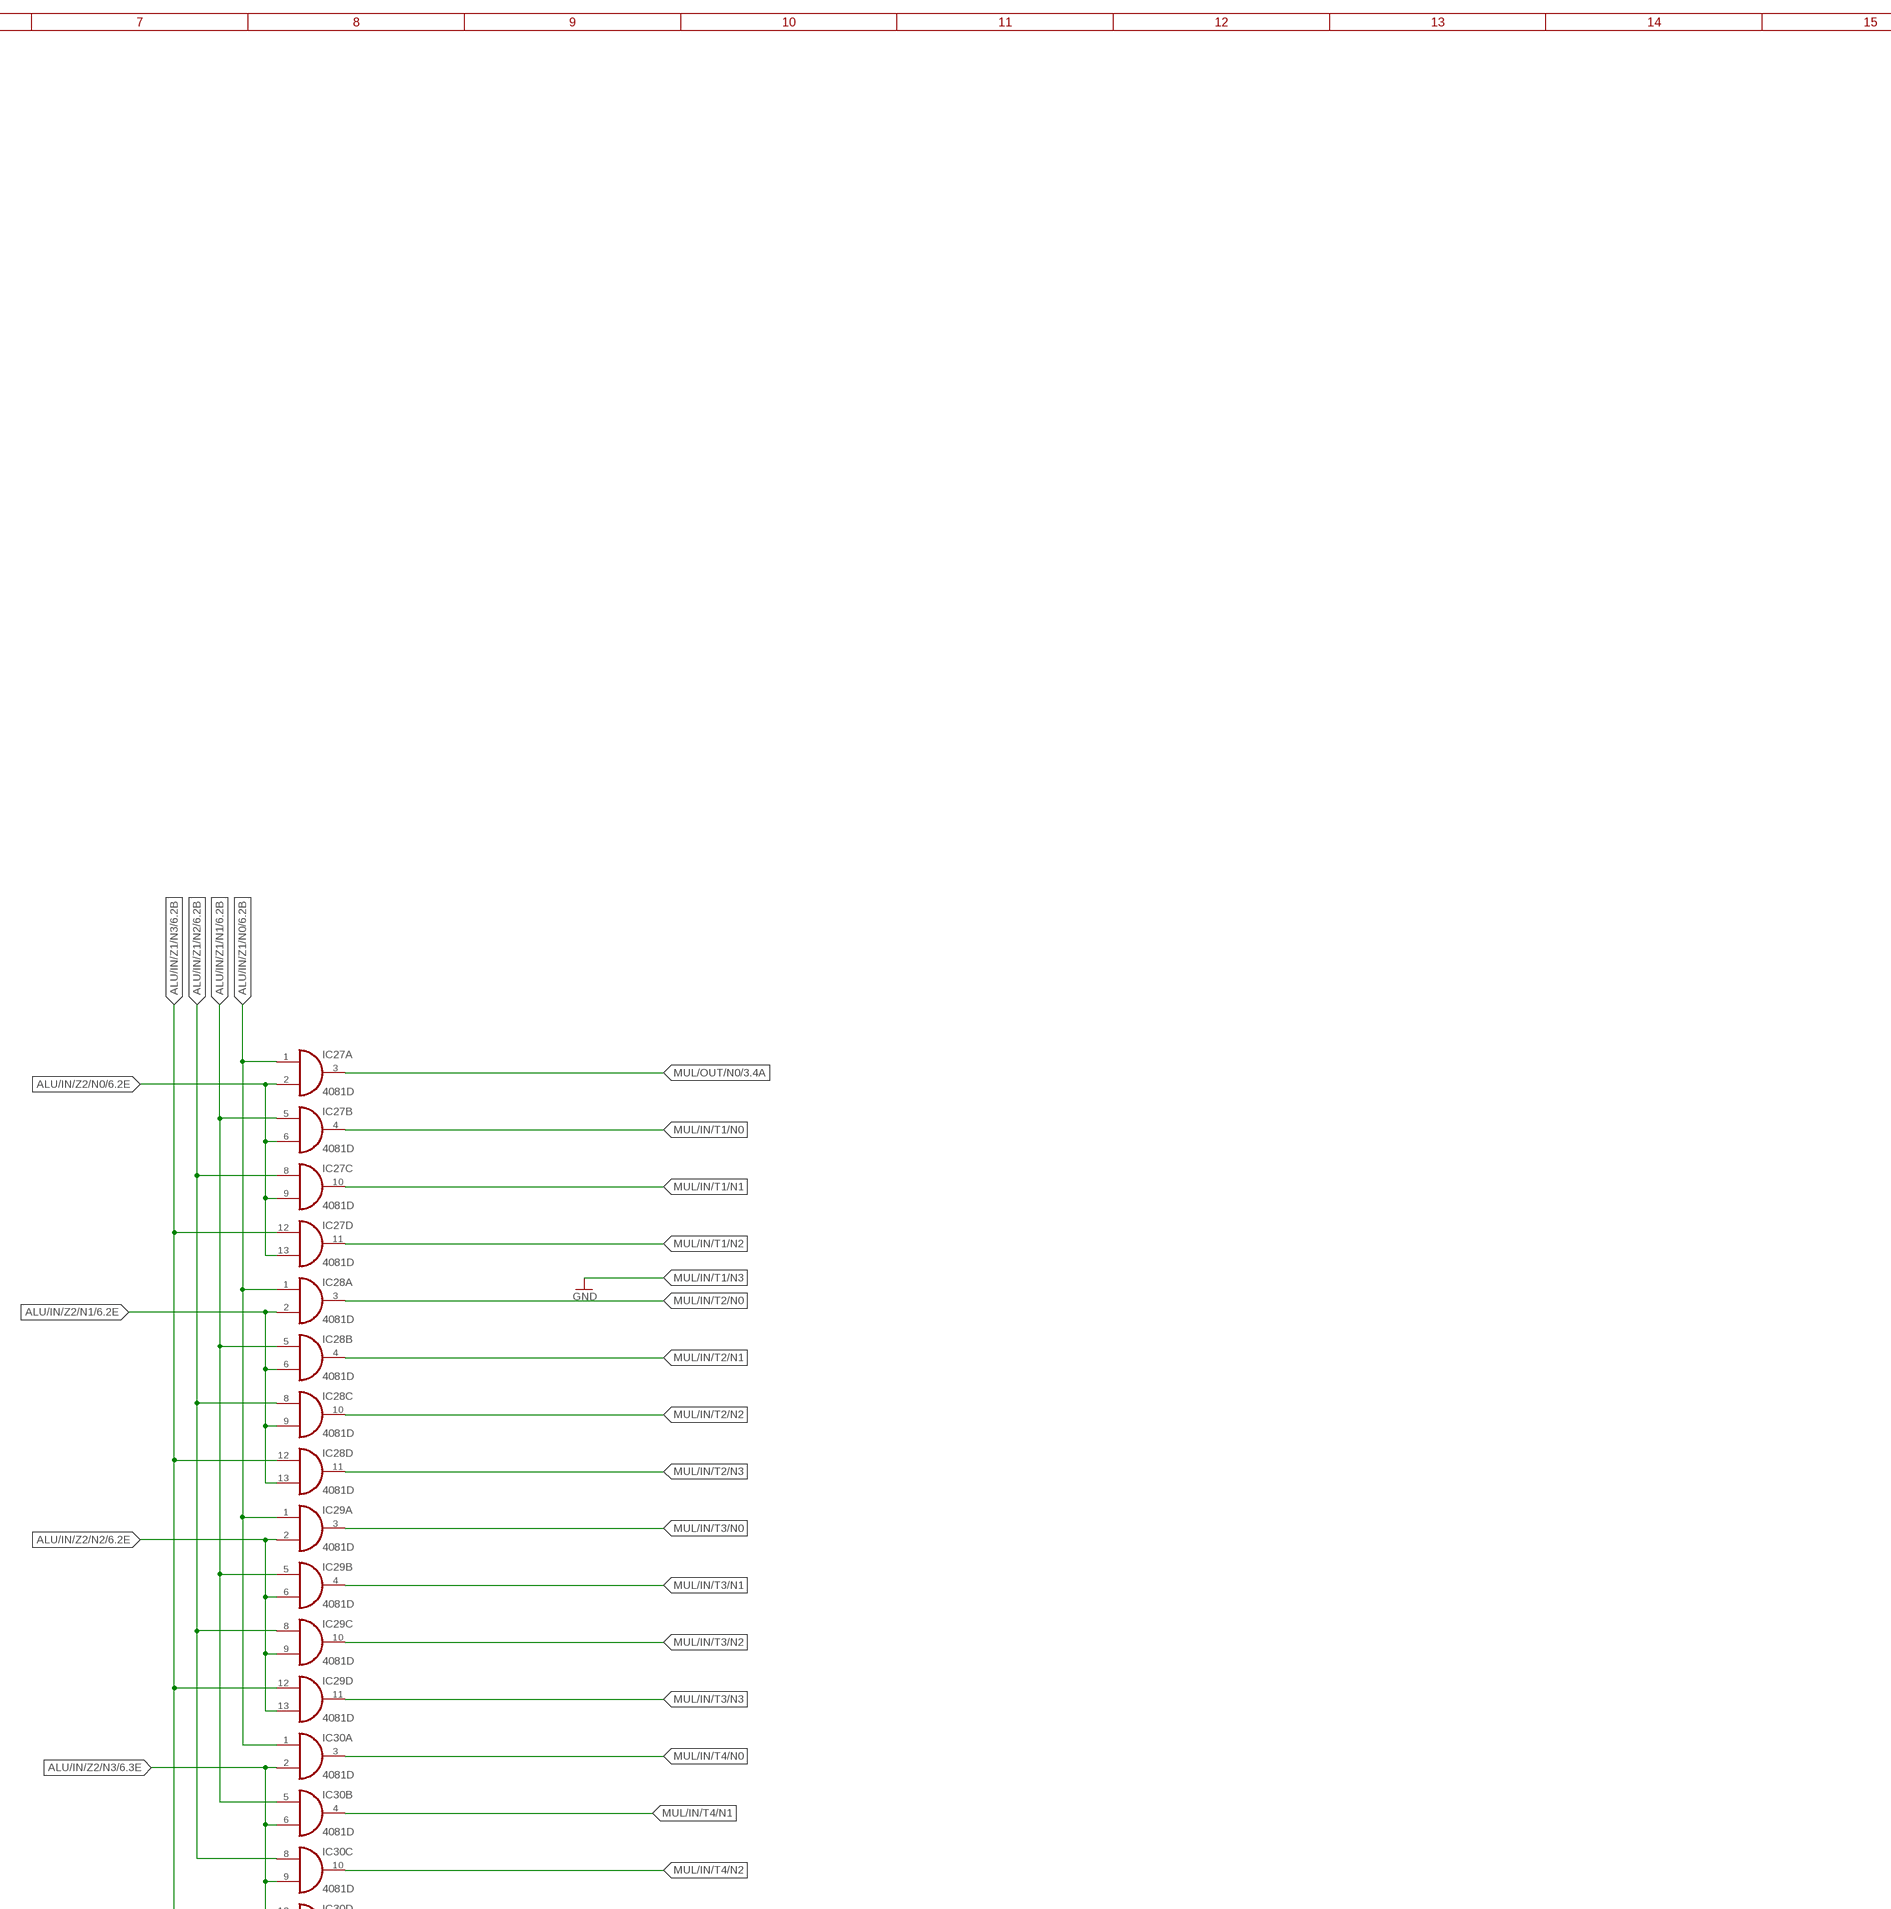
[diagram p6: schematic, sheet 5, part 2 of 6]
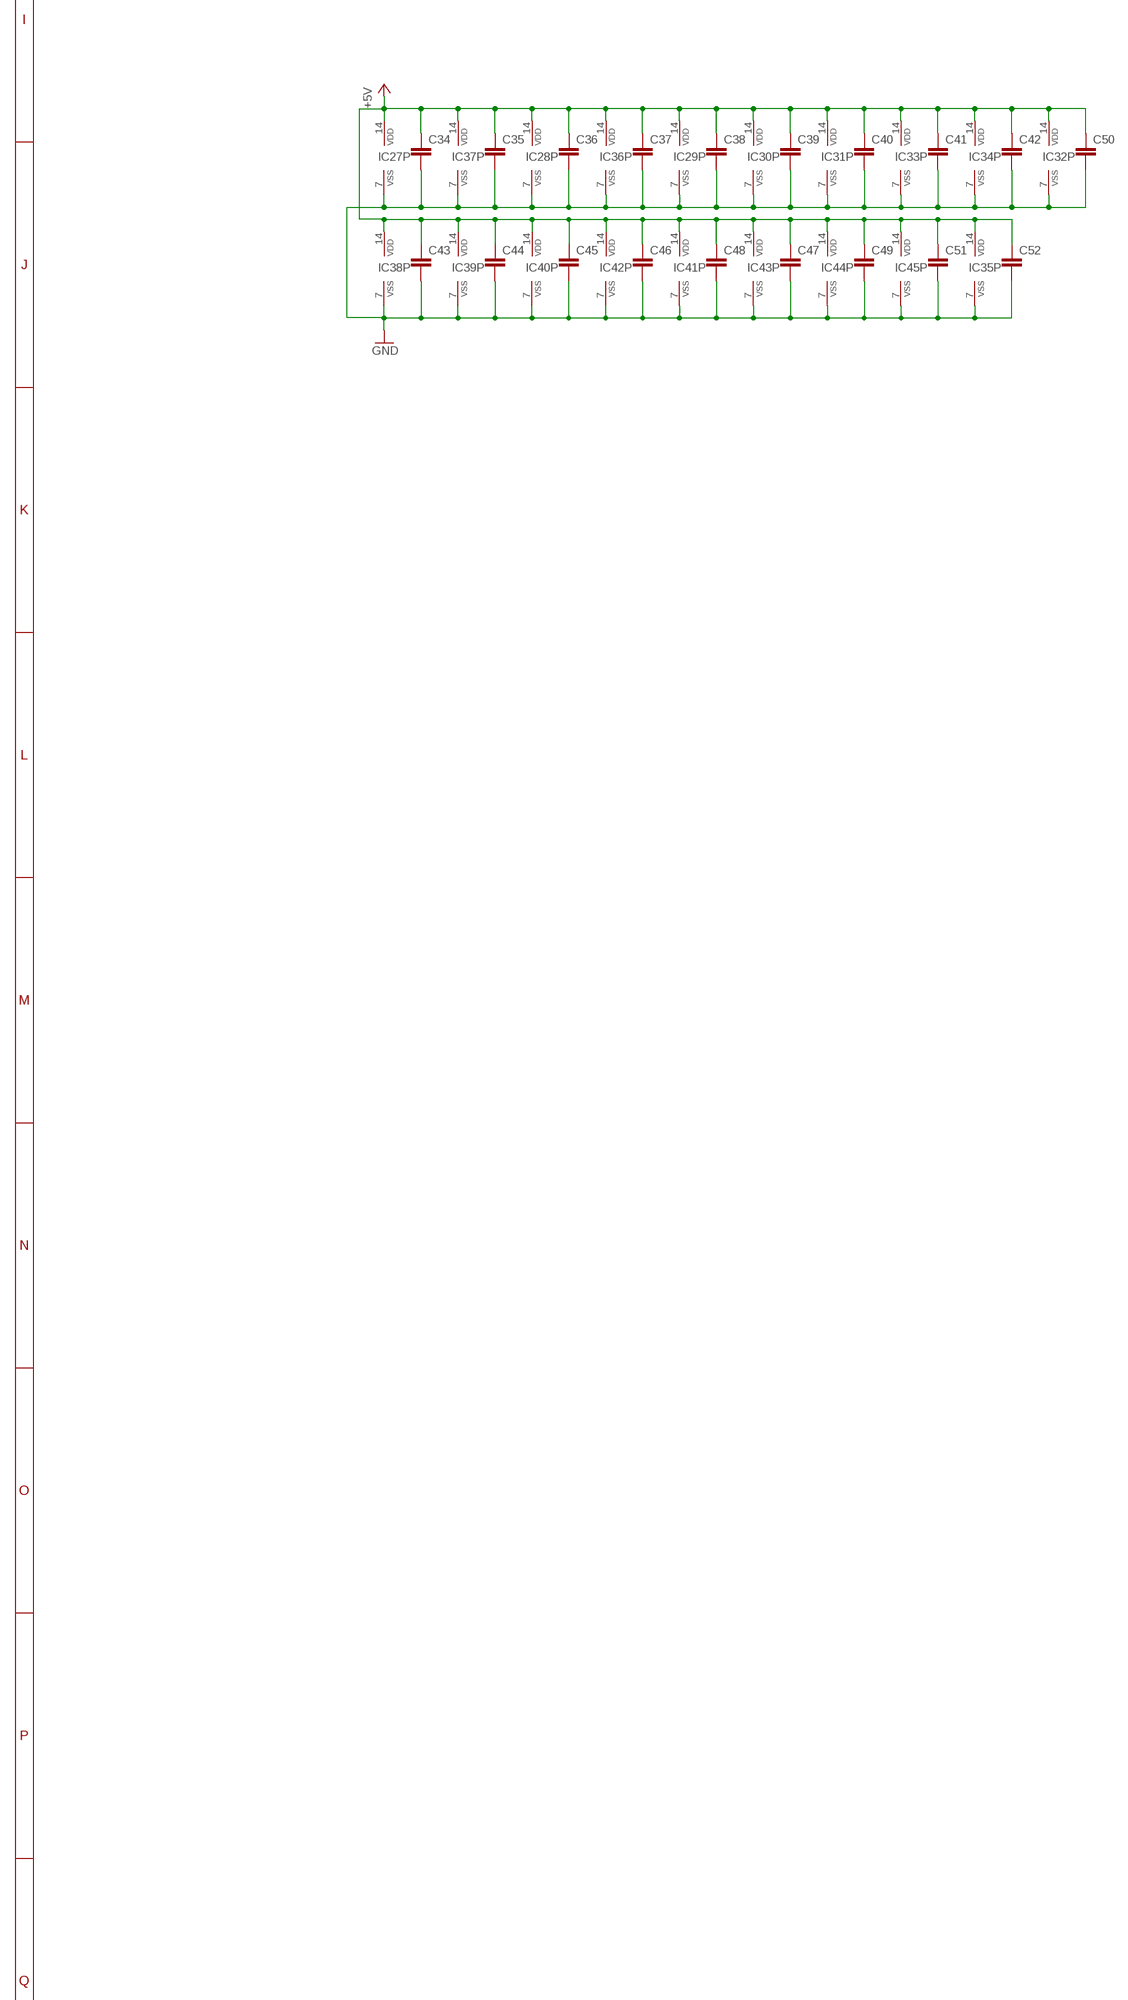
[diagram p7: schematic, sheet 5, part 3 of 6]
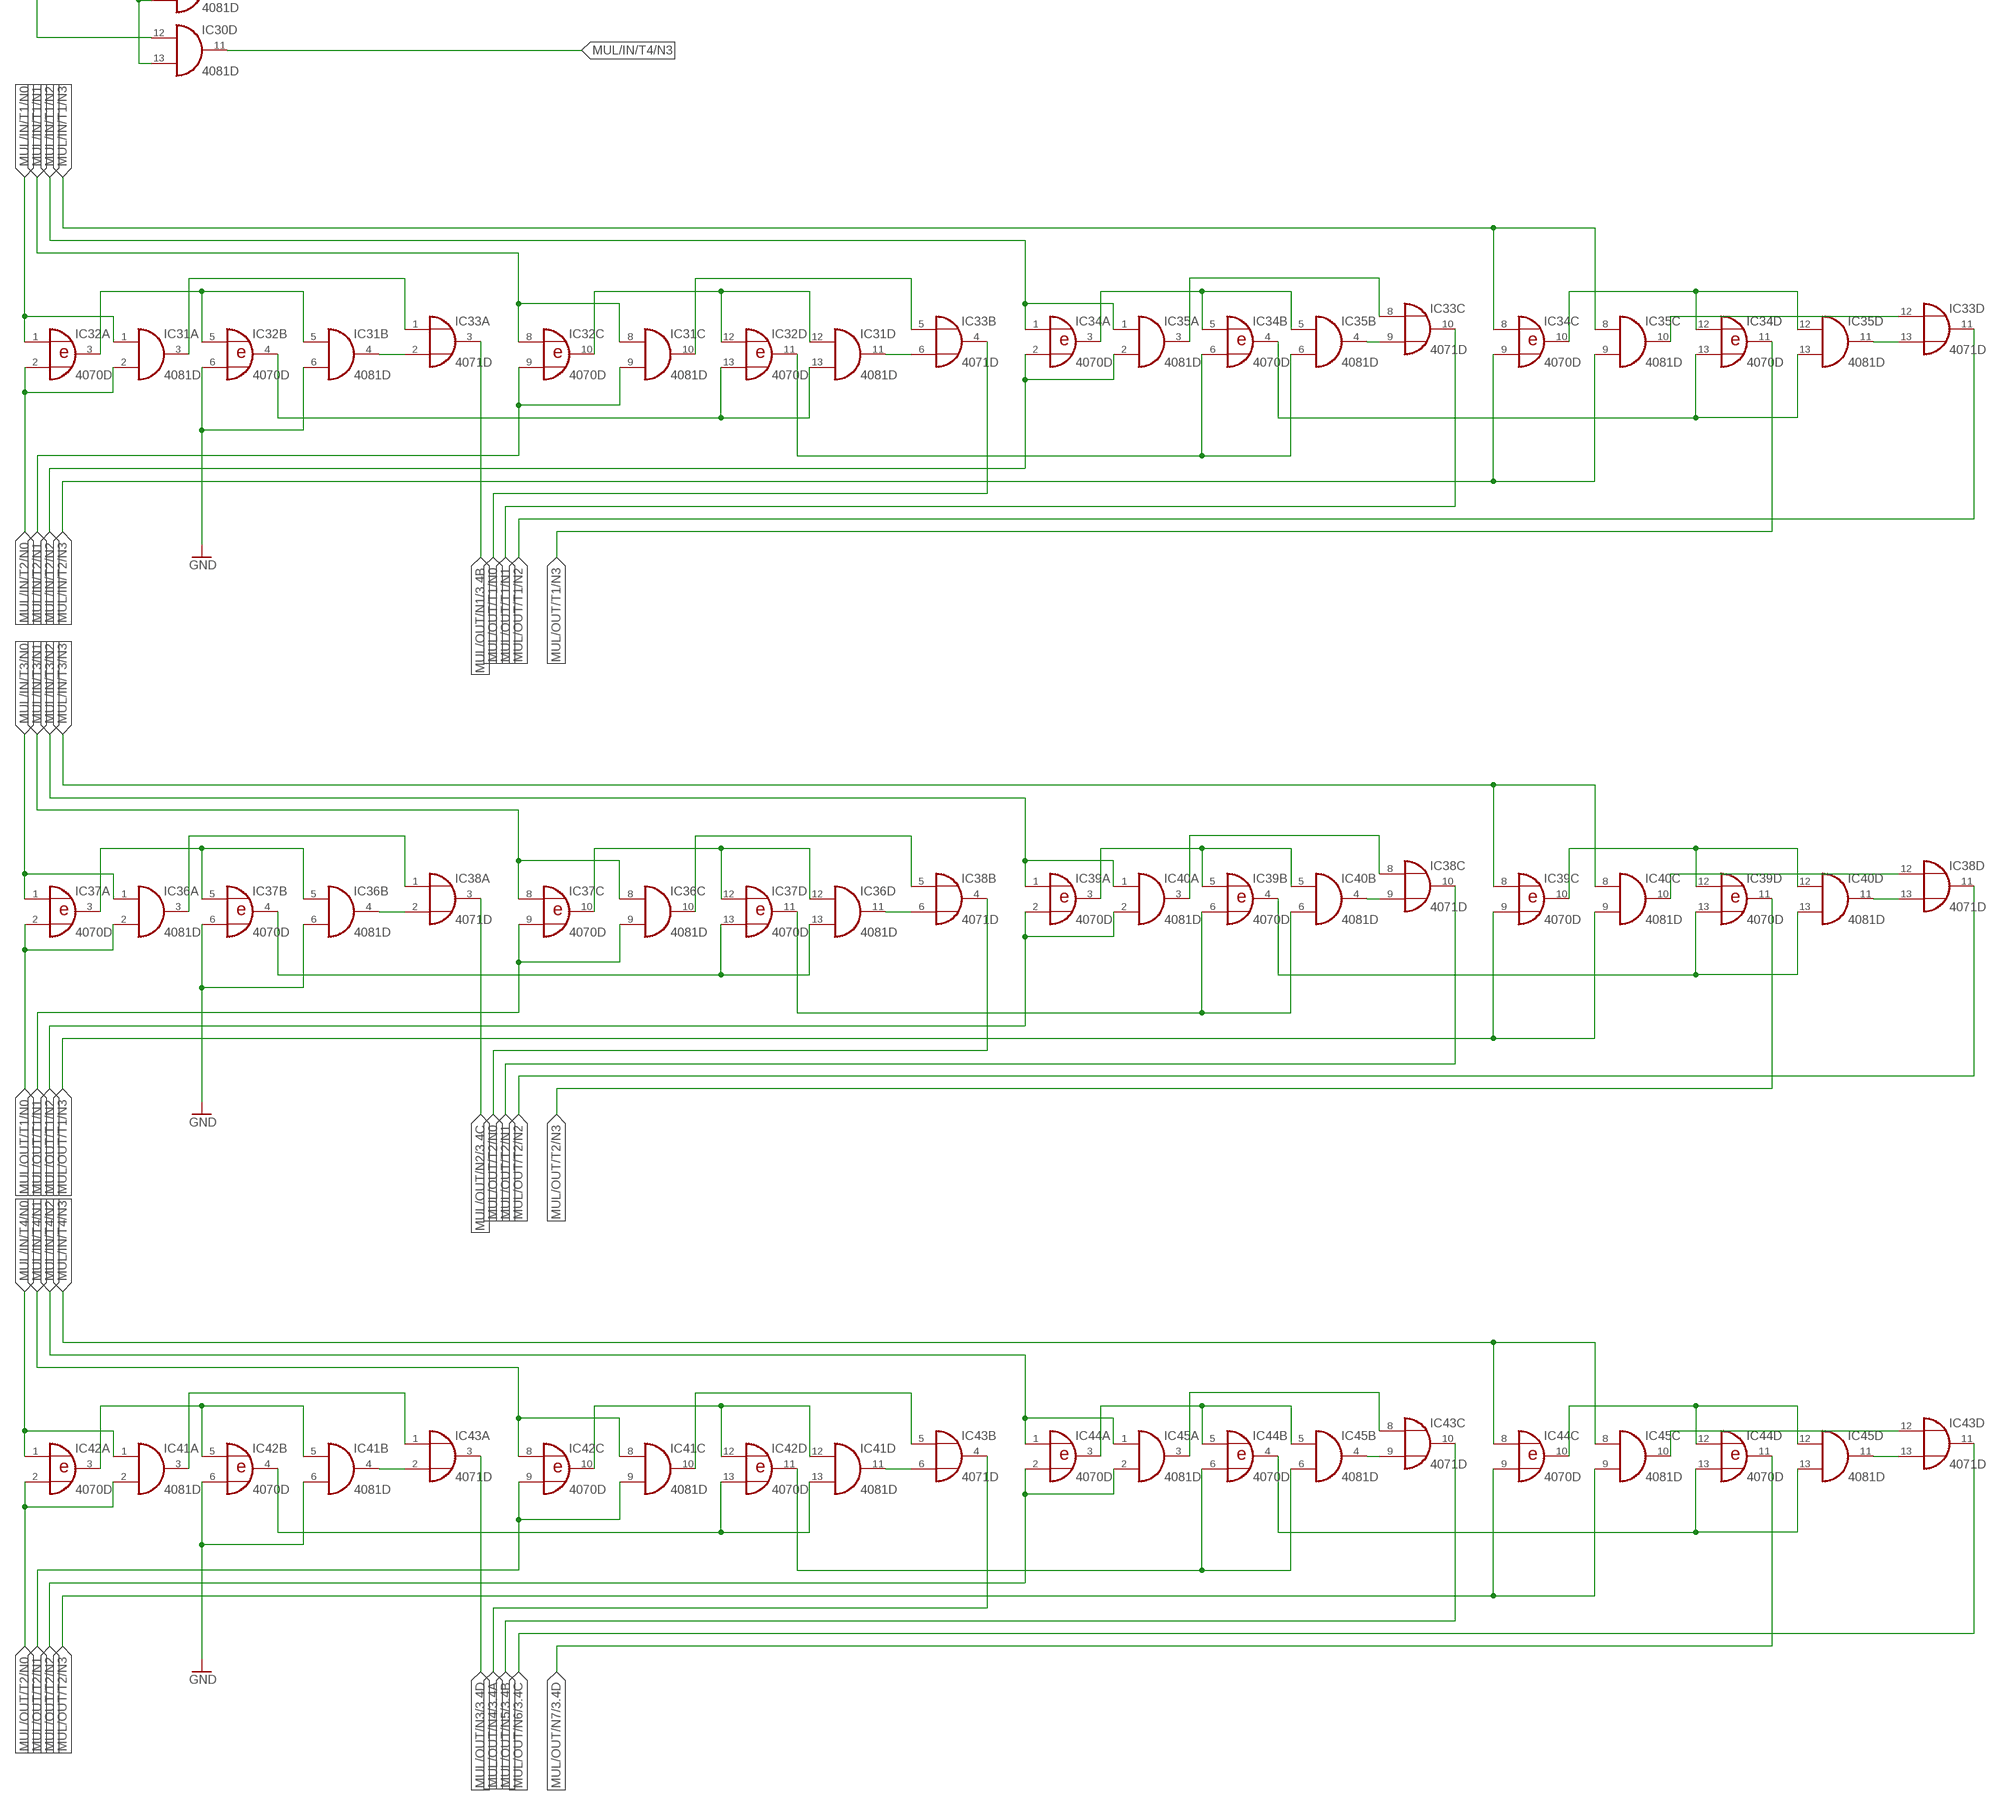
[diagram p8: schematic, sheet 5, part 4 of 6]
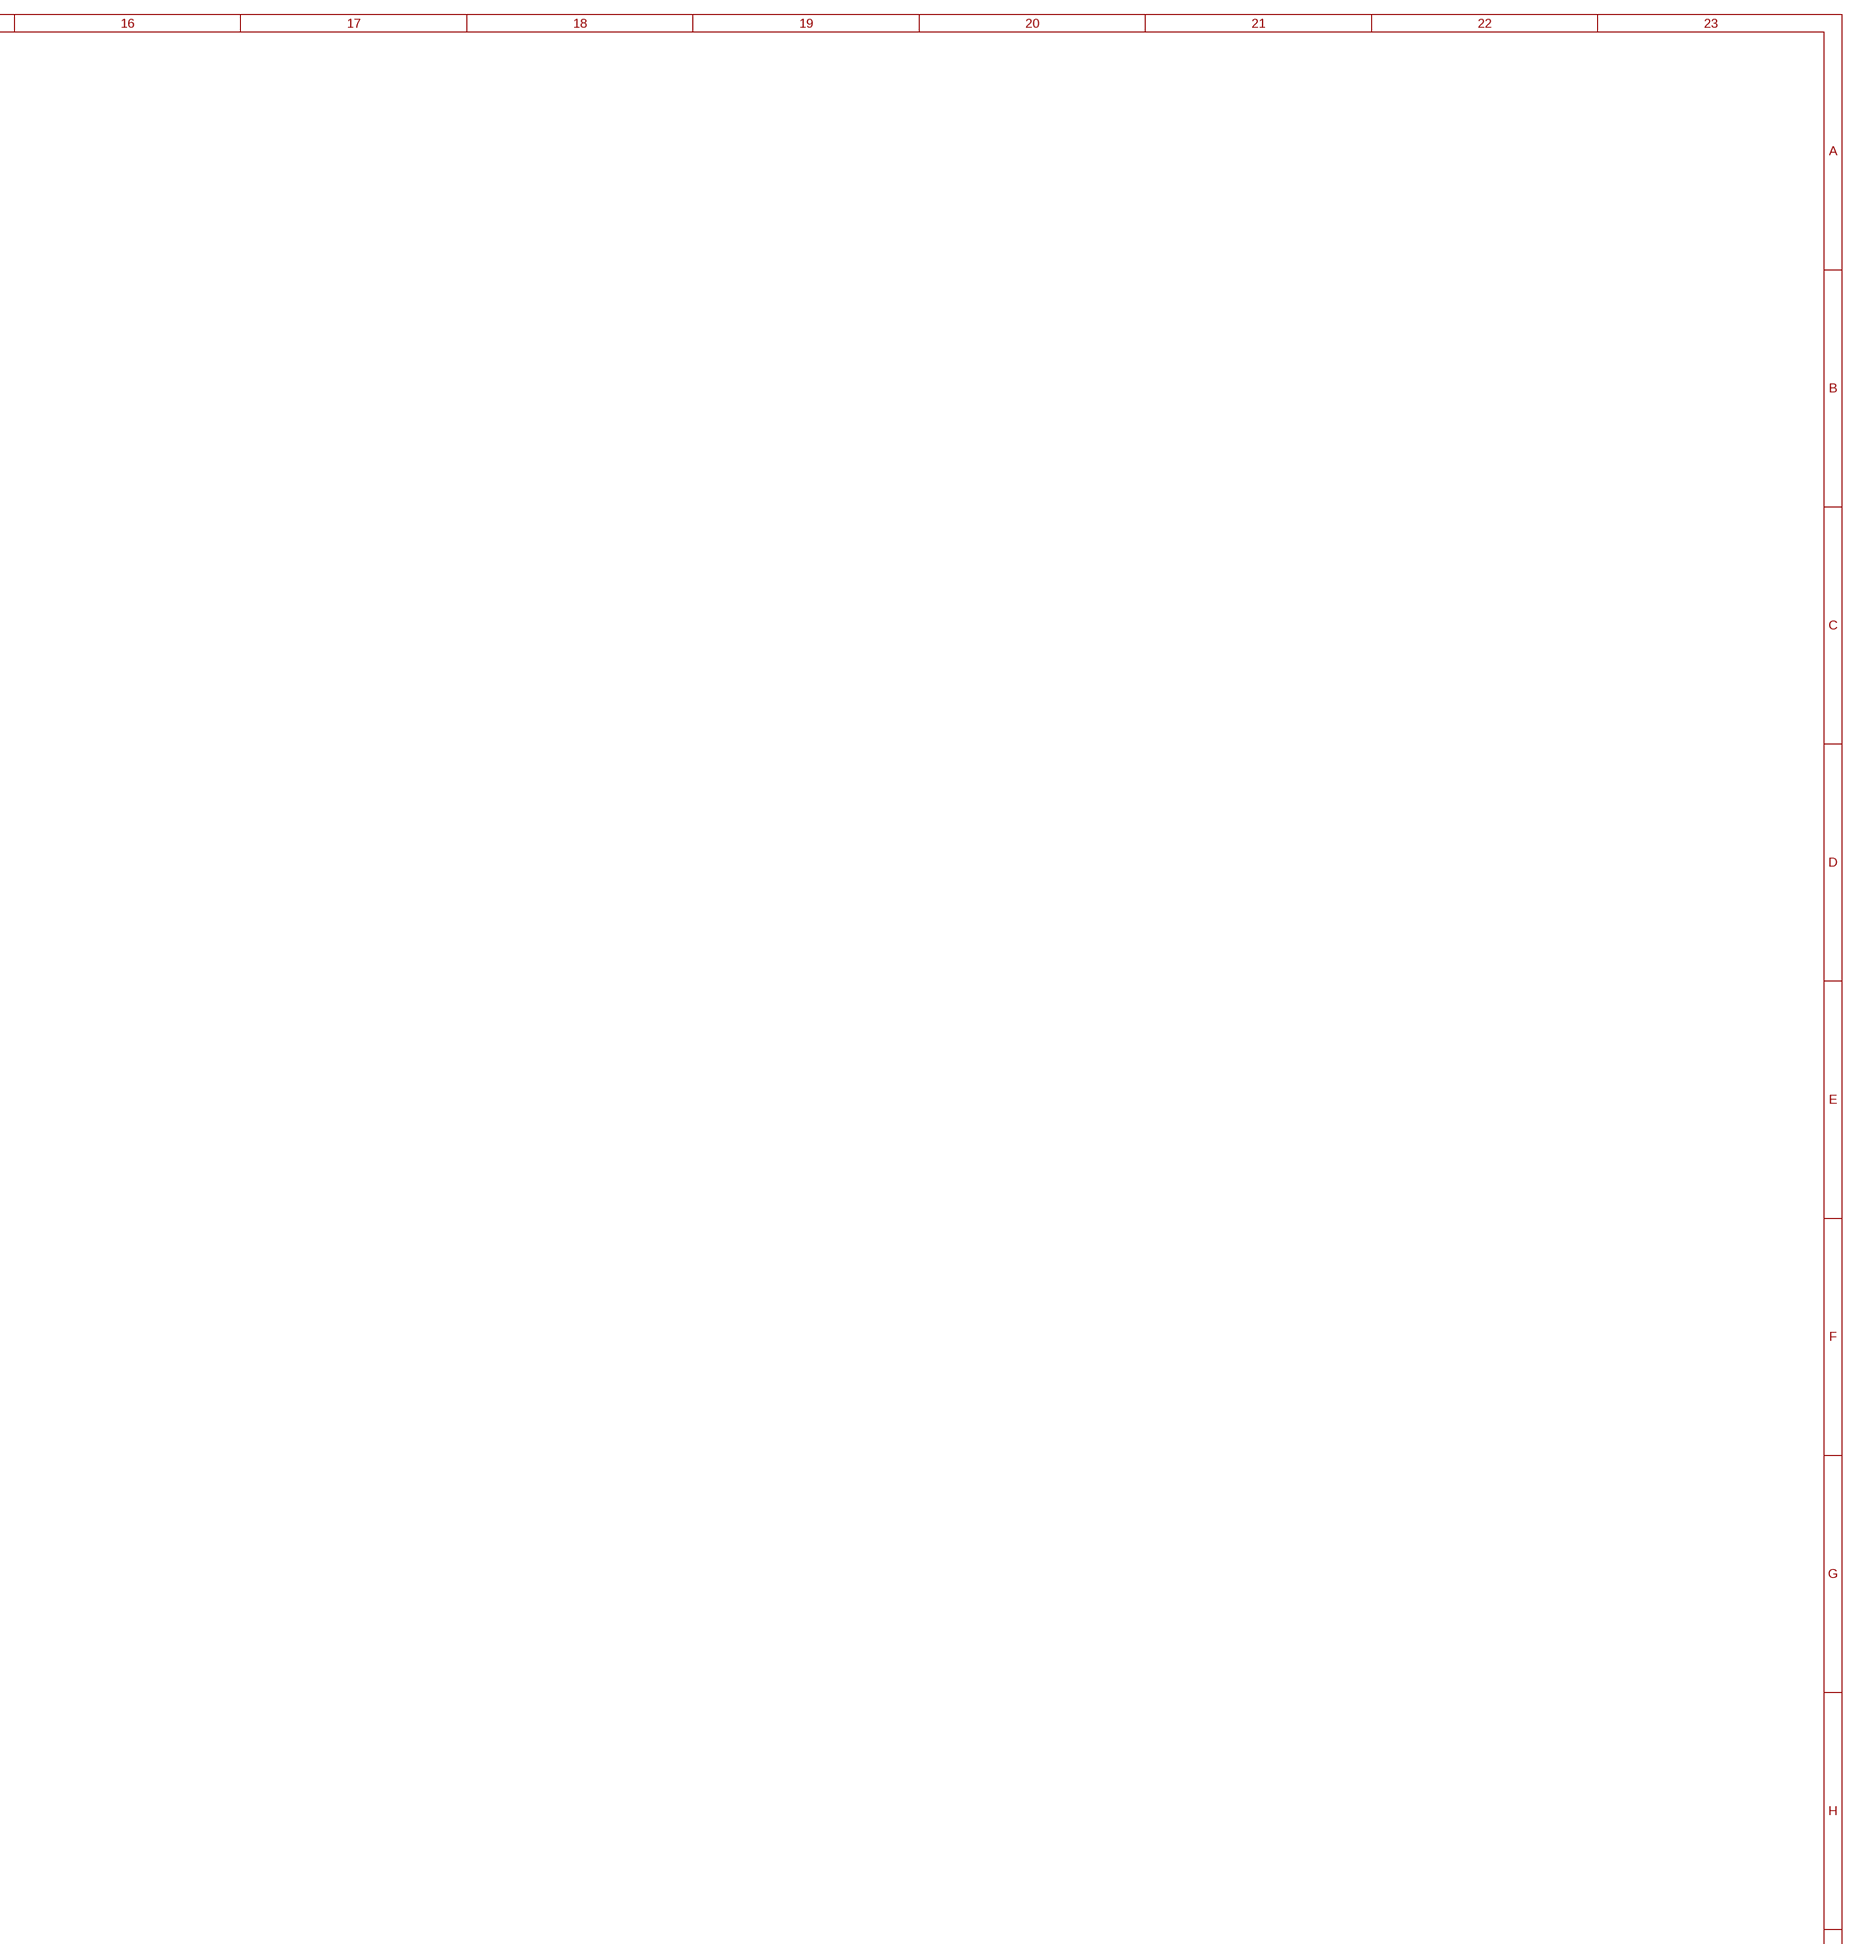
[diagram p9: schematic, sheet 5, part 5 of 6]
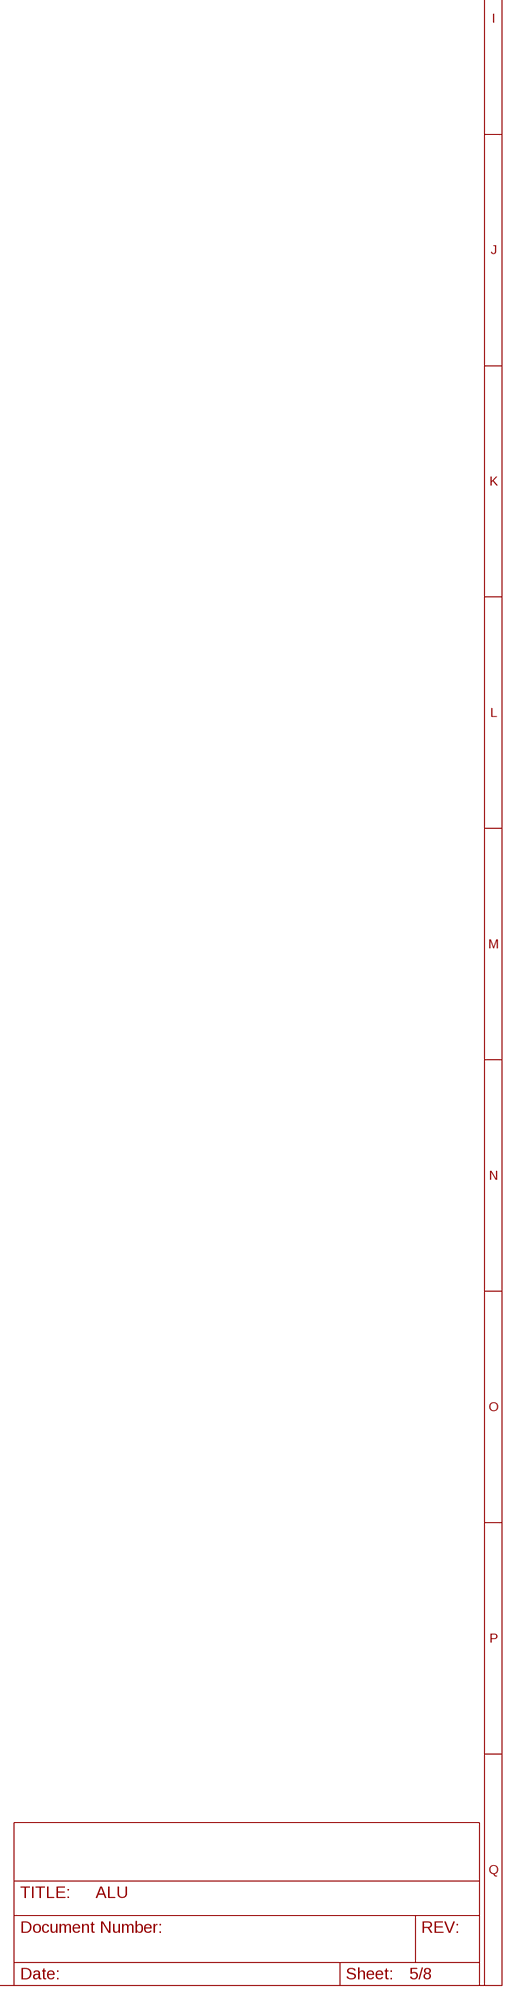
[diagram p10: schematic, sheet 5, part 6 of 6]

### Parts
C34  C-EUC0805  [C0805]
C35  C-EUC0805  [C0805]
C36  C-EUC0805  [C0805]
C37  C-EUC0805  [C0805]
C38  C-EUC0805  [C0805]
C39  C-EUC0805  [C0805]
C40  C-EUC0805  [C0805]
C41  C-EUC0805  [C0805]
C42  C-EUC0805  [C0805]
C43  C-EUC0805  [C0805]
C44  C-EUC0805  [C0805]
C45  C-EUC0805  [C0805]
C46  C-EUC0805  [C0805]
C47  C-EUC0805  [C0805]
C48  C-EUC0805  [C0805]
C49  C-EUC0805  [C0805]
C50  C-EUC0805  [C0805]
C51  C-EUC0805  [C0805]
C52  C-EUC0805  [C0805]
IC27  4081D  [SO14]
IC28  4081D  [SO14]
IC29  4081D  [SO14]
IC30  4081D  [SO14]
IC31  4081D  [SO14]
IC32  4070D  [SO14]
IC33  4071D  [SO14]
IC34  4070D  [SO14]
IC35  4081D  [SO14]
IC36  4081D  [SO14]
IC37  4070D  [SO14]
IC38  4071D  [SO14]
IC39  4070D  [SO14]
IC40  4081D  [SO14]
IC41  4081D  [SO14]
IC42  4070D  [SO14]
IC43  4071D  [SO14]
IC44  4070D  [SO14]
IC45  4081D  [SO14]

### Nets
+5V: C34.1 C35.1 C36.1 C37.1 C38.1 C39.1 C40.1 C41.1 C42.1 C43.1 C44.1 C45.1 C46.1 C47.1 C48.1 C49.1 C50.1 C51.1 C52.1 IC27.14(P:VDD) IC28.14(P:VDD) IC29.14(P:VDD) IC30.14(P:VDD) IC31.14(P:VDD) IC32.14(P:VDD) IC33.14(P:VDD) IC34.14(P:VDD) IC35.14(P:VDD) IC36.14(P:VDD) IC37.14(P:VDD) IC38.14(P:VDD) IC39.14(P:VDD) IC40.14(P:VDD) IC41.14(P:VDD) IC42.14(P:VDD) IC43.14(P:VDD) IC44.14(P:VDD) IC45.14(P:VDD) ; also sheet 1,2,3,4,6,7,8
ALU/IN/Z1/N0: IC27.1(A:I0) IC28.1(A:I0) IC29.1(A:I0) IC30.1(A:I0) ; also sheet 1,2,4,6,7
ALU/IN/Z1/N1: IC27.5(B:I0) IC28.5(B:I0) IC29.5(B:I0) IC30.5(B:I0) ; also sheet 1,2,4,6,7
ALU/IN/Z1/N2: IC27.8(C:I0) IC28.8(C:I0) IC29.8(C:I0) IC30.8(C:I0) ; also sheet 1,2,4,6,7
ALU/IN/Z1/N3: IC27.12(D:I0) IC28.12(D:I0) IC29.12(D:I0) IC30.12(D:I0) ; also sheet 1,2,4,6,7
ALU/IN/Z2/N0: IC27.2(A:I1) IC27.6(B:I1) IC27.9(C:I1) IC27.13(D:I1) ; also sheet 1,4,6,7
ALU/IN/Z2/N1: IC28.2(A:I1) IC28.6(B:I1) IC28.9(C:I1) IC28.13(D:I1) ; also sheet 1,4,6,7
ALU/IN/Z2/N2: IC29.2(A:I1) IC29.6(B:I1) IC29.9(C:I1) IC29.13(D:I1) ; also sheet 1,4,6,7
ALU/IN/Z2/N3: IC30.2(A:I1) IC30.6(B:I1) IC30.9(C:I1) IC30.13(D:I1) ; also sheet 1,4,6,7
GND: C34.2 C35.2 C36.2 C37.2 C38.2 C39.2 C40.2 C41.2 C42.2 C43.2 C44.2 C45.2 C46.2 C47.2 C48.2 C49.2 C50.2 C51.2 C52.2 IC27.7(P:VSS) IC28.7(P:VSS) IC29.7(P:VSS) IC30.7(P:VSS) IC31.6(B:I1) IC31.7(P:VSS) IC32.6(B:I1) IC32.7(P:VSS) IC33.7(P:VSS) IC34.7(P:VSS) IC35.7(P:VSS) IC36.6(B:I1) IC36.7(P:VSS) IC37.6(B:I1) IC37.7(P:VSS) IC38.7(P:VSS) IC39.7(P:VSS) IC40.7(P:VSS) IC41.6(B:I1) IC41.7(P:VSS) IC42.6(B:I1) IC42.7(P:VSS) IC43.7(P:VSS) IC44.7(P:VSS) IC45.7(P:VSS) ; also sheet 1,2,3,4,6,7,8
MUL/IN/T1/N0: IC27.4(B:O) IC31.1(A:I0) IC32.1(A:I0)
MUL/IN/T1/N1: IC27.10(C:O) IC31.8(C:I0) IC32.8(C:I0)
MUL/IN/T1/N2: IC27.11(D:O) IC34.1(A:I0) IC35.1(A:I0)
MUL/IN/T1/N3: IC34.8(C:I0) IC35.8(C:I0) ; supply symbol labelled GND
MUL/IN/T2/N0: IC28.3(A:O) IC31.2(A:I1) IC32.2(A:I1)
MUL/IN/T2/N1: IC28.4(B:O) IC31.9(C:I1) IC32.9(C:I1)
MUL/IN/T2/N2: IC28.10(C:O) IC34.2(A:I1) IC35.2(A:I1)
MUL/IN/T2/N3: IC28.11(D:O) IC34.9(C:I1) IC35.9(C:I1)
MUL/IN/T3/N0: IC29.3(A:O) IC36.1(A:I0) IC37.1(A:I0)
MUL/IN/T3/N1: IC29.4(B:O) IC36.8(C:I0) IC37.8(C:I0)
MUL/IN/T3/N2: IC29.10(C:O) IC39.1(A:I0) IC40.1(A:I0)
MUL/IN/T3/N3: IC29.11(D:O) IC39.8(C:I0) IC40.8(C:I0)
MUL/IN/T4/N0: IC30.3(A:O) IC41.1(A:I0) IC42.1(A:I0)
MUL/IN/T4/N1: IC30.4(B:O) IC41.8(C:I0) IC42.8(C:I0)
MUL/IN/T4/N2: IC30.10(C:O) IC44.1(A:I0) IC45.1(A:I0)
MUL/IN/T4/N3: IC30.11(D:O) IC44.8(C:I0) IC45.8(C:I0)
MUL/OUT/N0: IC27.3(A:O) ; also sheet 3
MUL/OUT/N1: IC33.3(A:O) ; also sheet 3
MUL/OUT/N2: IC38.3(A:O) ; also sheet 3
MUL/OUT/N3: IC43.3(A:O) ; also sheet 3
MUL/OUT/N4: IC43.4(B:O) ; also sheet 3
MUL/OUT/N5: IC43.10(C:O) ; also sheet 3
MUL/OUT/N6: IC43.11(D:O) ; also sheet 3
MUL/OUT/N7: IC44.11(D:O) ; also sheet 3
MUL/OUT/T1/N0: IC33.4(B:O) IC36.2(A:I1) IC37.2(A:I1)
MUL/OUT/T1/N1: IC33.10(C:O) IC36.9(C:I1) IC37.9(C:I1)
MUL/OUT/T1/N2: IC33.11(D:O) IC39.2(A:I1) IC40.2(A:I1)
MUL/OUT/T1/N3: IC34.11(D:O) IC39.9(C:I1) IC40.9(C:I1)
MUL/OUT/T2/N0: IC38.4(B:O) IC41.2(A:I1) IC42.2(A:I1)
MUL/OUT/T2/N1: IC38.10(C:O) IC41.9(C:I1) IC42.9(C:I1)
MUL/OUT/T2/N2: IC38.11(D:O) IC44.2(A:I1) IC45.2(A:I1)
MUL/OUT/T2/N3: IC39.11(D:O) IC44.9(C:I1) IC45.9(C:I1)
N$74: IC31.5(B:I0) IC32.3(A:O) IC32.5(B:I0)
N$75: IC31.3(A:O) IC33.1(A:I0)
N$76: IC31.4(B:O) IC33.2(A:I1)
N$77: IC31.13(D:I1) IC32.4(B:O) IC32.13(D:I1)
N$78: IC32.11(D:O) IC34.6(B:I1) IC35.6(B:I1)
N$79: IC31.12(D:I0) IC32.10(C:O) IC32.12(D:I0)
N$80: IC31.10(C:O) IC33.5(B:I0)
N$81: IC31.11(D:O) IC33.6(B:I1)
N$82: IC34.3(A:O) IC34.5(B:I0) IC35.5(B:I0)
N$83: IC34.4(B:O) IC34.13(D:I1) IC35.13(D:I1)
N$84: IC33.9(C:I1) IC35.4(B:O)
N$85: IC33.8(C:I0) IC35.3(A:O)
N$86: IC34.10(C:O) IC34.12(D:I0) IC35.12(D:I0)
N$87: IC33.12(D:I0) IC35.10(C:O)
N$88: IC33.13(D:I1) IC35.11(D:O)
N$89: IC36.5(B:I0) IC37.3(A:O) IC37.5(B:I0)
N$90: IC36.3(A:O) IC38.1(A:I0)
N$91: IC36.4(B:O) IC38.2(A:I1)
N$92: IC36.13(D:I1) IC37.4(B:O) IC37.13(D:I1)
N$93: IC37.11(D:O) IC39.6(B:I1) IC40.6(B:I1)
N$94: IC36.12(D:I0) IC37.10(C:O) IC37.12(D:I0)
N$95: IC36.10(C:O) IC38.5(B:I0)
N$96: IC36.11(D:O) IC38.6(B:I1)
N$97: IC39.3(A:O) IC39.5(B:I0) IC40.5(B:I0)
N$98: IC39.4(B:O) IC39.13(D:I1) IC40.13(D:I1)
N$99: IC38.9(C:I1) IC40.4(B:O)
N$100: IC38.8(C:I0) IC40.3(A:O)
N$101: IC39.10(C:O) IC39.12(D:I0) IC40.12(D:I0)
N$102: IC38.12(D:I0) IC40.10(C:O)
N$103: IC38.13(D:I1) IC40.11(D:O)
N$104: IC41.5(B:I0) IC42.3(A:O) IC42.5(B:I0)
N$105: IC41.3(A:O) IC43.1(A:I0)
N$107: IC41.4(B:O) IC43.2(A:I1)
N$108: IC41.13(D:I1) IC42.4(B:O) IC42.13(D:I1)
N$109: IC42.11(D:O) IC44.6(B:I1) IC45.6(B:I1)
N$110: IC41.12(D:I0) IC42.10(C:O) IC42.12(D:I0)
N$111: IC41.10(C:O) IC43.5(B:I0)
N$112: IC41.11(D:O) IC43.6(B:I1)
N$113: IC44.3(A:O) IC44.5(B:I0) IC45.5(B:I0)
N$114: IC44.4(B:O) IC44.13(D:I1) IC45.13(D:I1)
N$115: IC43.9(C:I1) IC45.4(B:O)
N$116: IC43.8(C:I0) IC45.3(A:O)
N$117: IC44.10(C:O) IC44.12(D:I0) IC45.12(D:I0)
N$118: IC43.12(D:I0) IC45.10(C:O)
N$119: IC43.13(D:I1) IC45.11(D:O)

## Sheet 6 of 8: subtrahierer
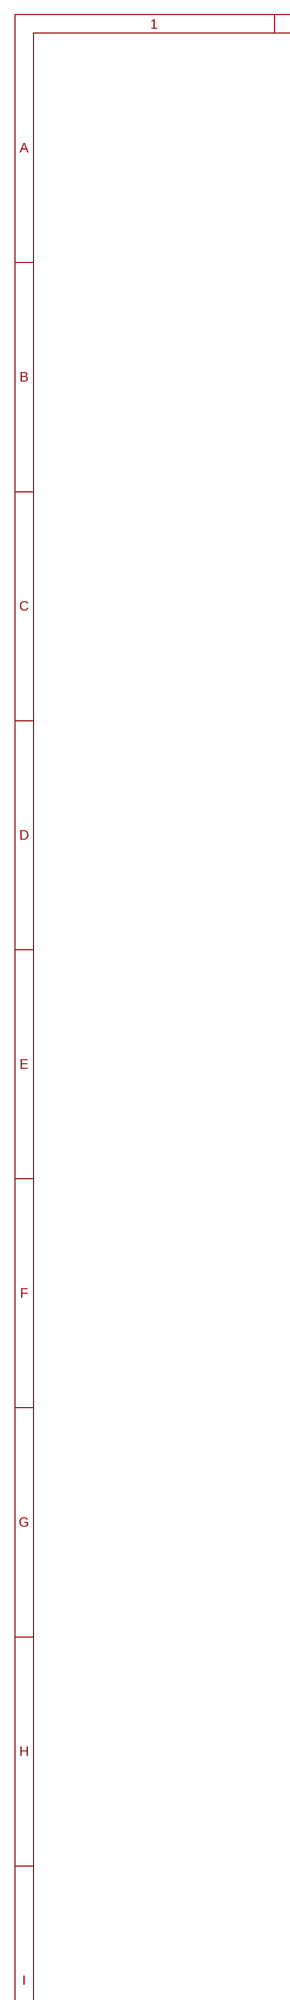
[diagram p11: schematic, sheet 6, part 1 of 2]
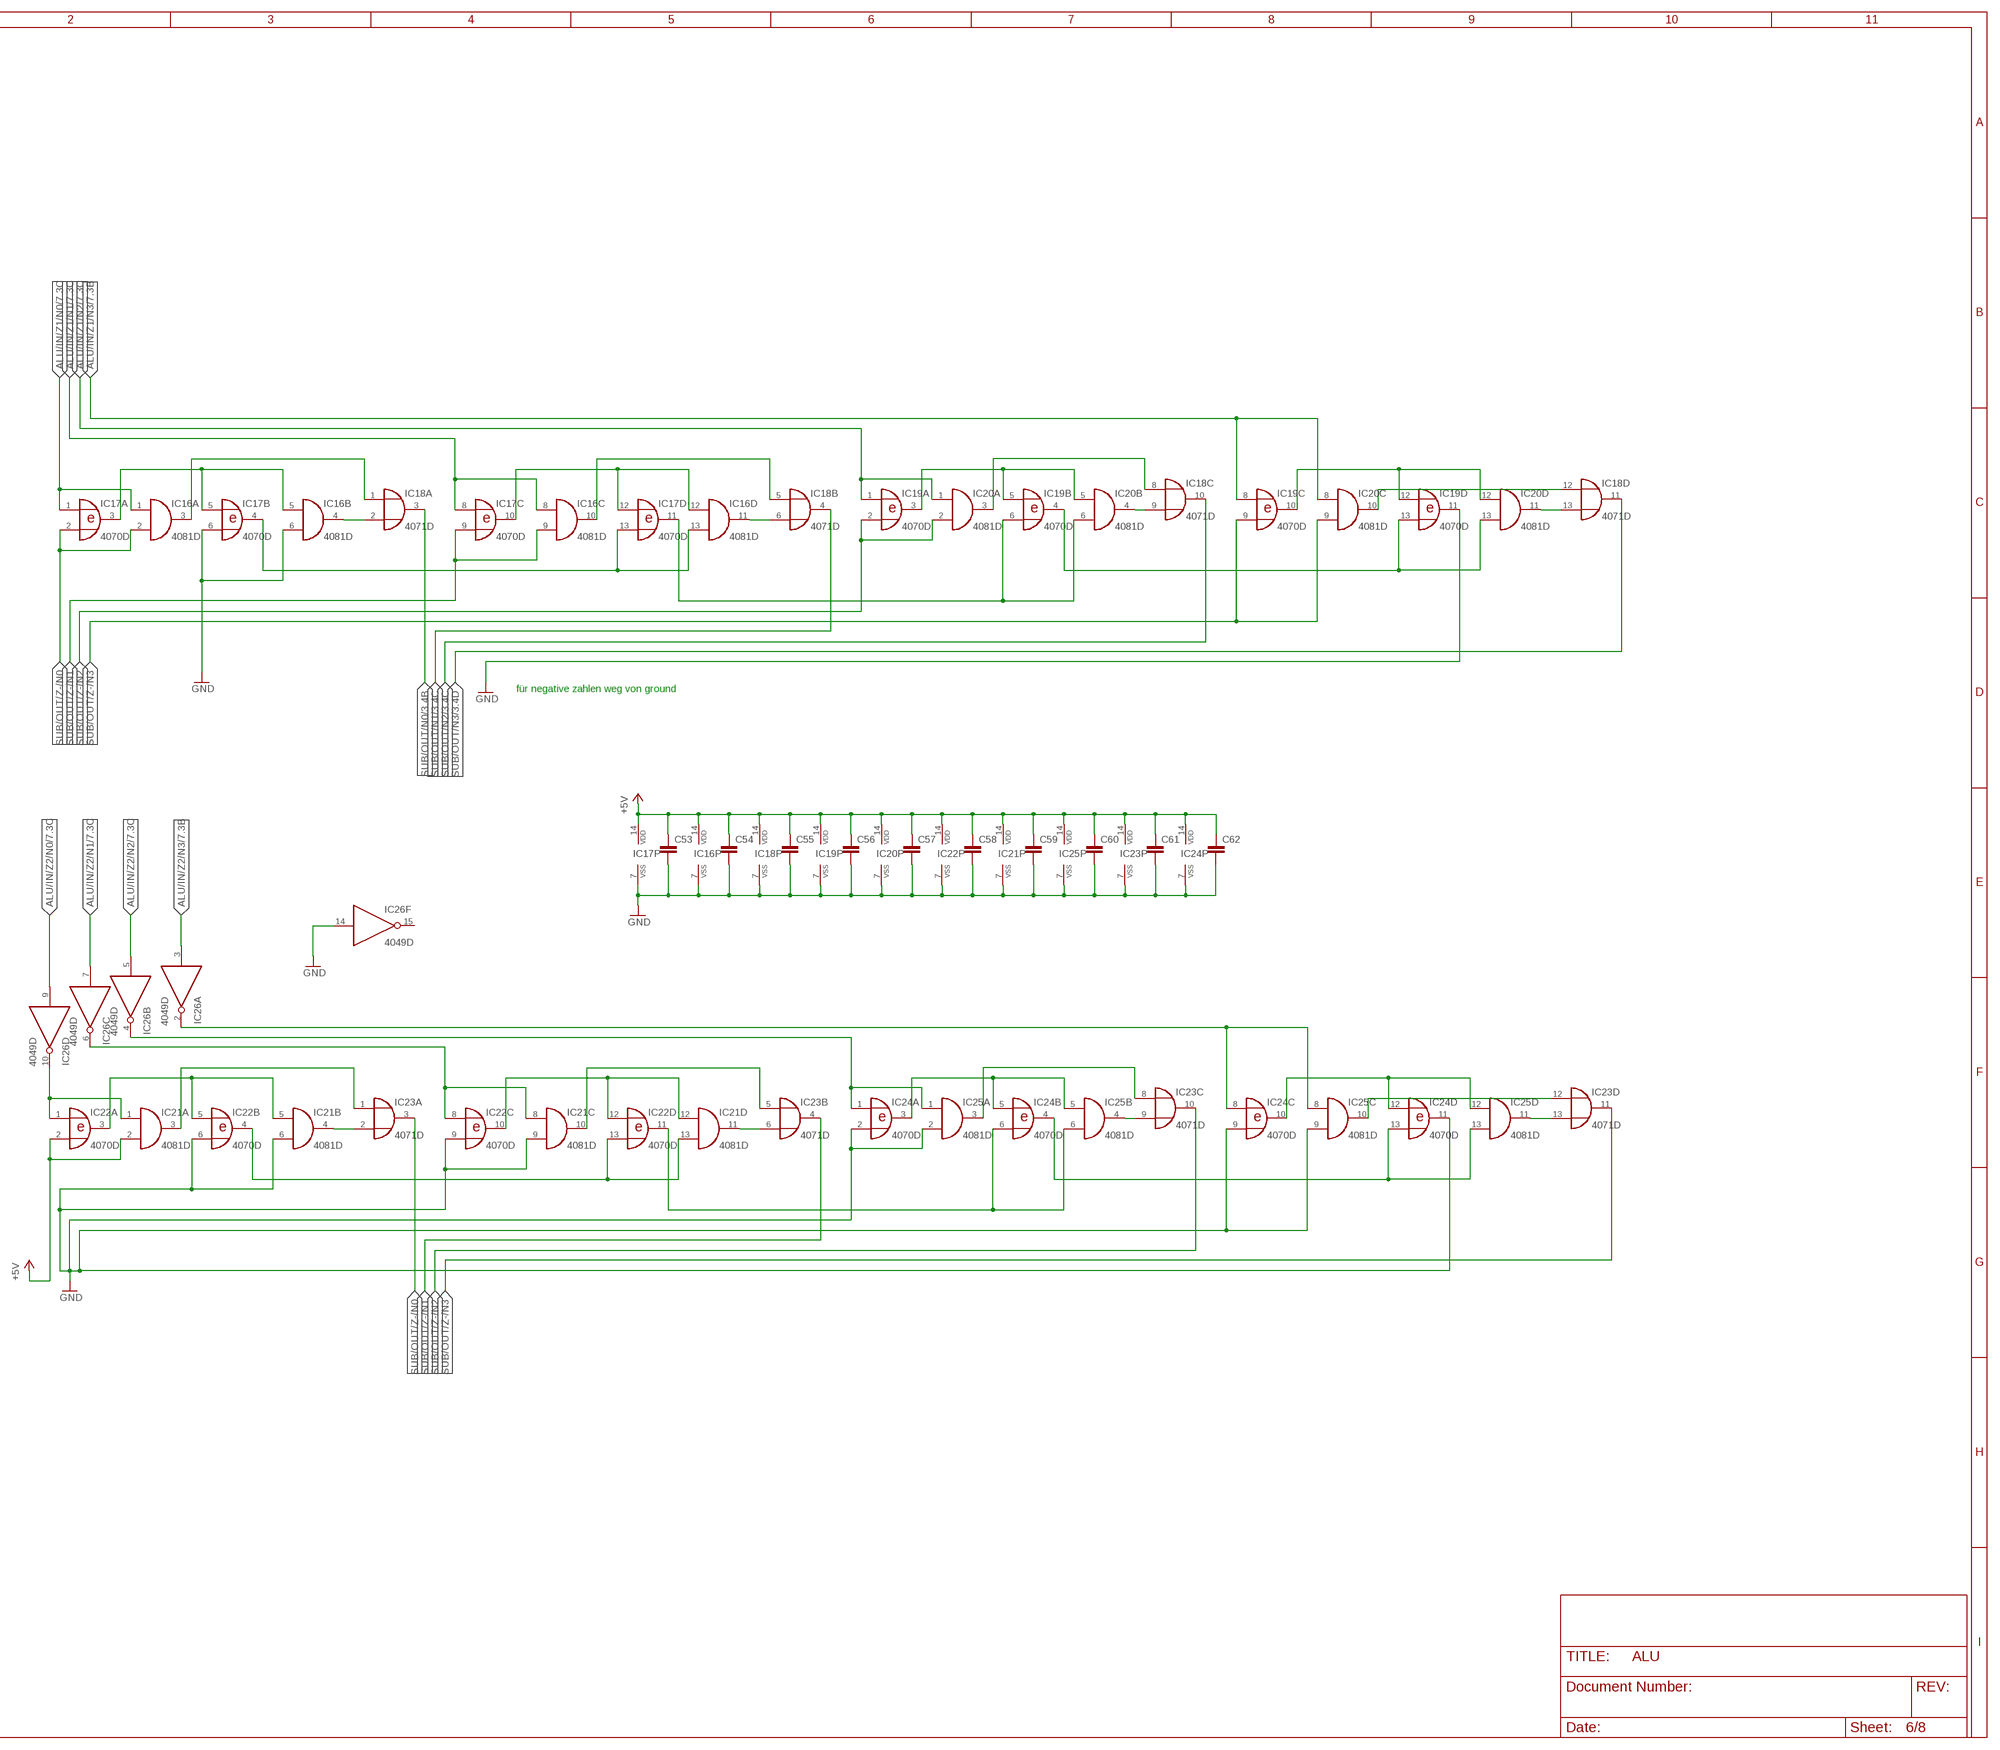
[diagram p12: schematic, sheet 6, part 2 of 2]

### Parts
C53  C-EUC0805  [C0805]
C54  C-EUC0805  [C0805]
C55  C-EUC0805  [C0805]
C56  C-EUC0805  [C0805]
C57  C-EUC0805  [C0805]
C58  C-EUC0805  [C0805]
C59  C-EUC0805  [C0805]
C60  C-EUC0805  [C0805]
C61  C-EUC0805  [C0805]
C62  C-EUC0805  [C0805]
IC16  4081D  [SO14]
IC17  4070D  [SO14]
IC18  4071D  [SO14]
IC19  4070D  [SO14]
IC20  4081D  [SO14]
IC21  4081D  [SO14]
IC22  4070D  [SO14]
IC23  4071D  [SO14]
IC24  4070D  [SO14]
IC25  4081D  [SO14]

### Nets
+5V: C53.1 C54.1 C55.1 C56.1 C57.1 C58.1 C59.1 C60.1 C61.1 C62.1 IC16.14(P:VDD) IC17.14(P:VDD) IC18.14(P:VDD) IC19.14(P:VDD) IC20.14(P:VDD) IC21.2(A:I1) IC21.14(P:VDD) IC22.2(A:I1) IC22.14(P:VDD) IC23.14(P:VDD) IC24.14(P:VDD) IC25.14(P:VDD) ; also sheet 1,2,3,4,5,7,8
ALU/IN/Z1/N0: IC16.1(A:I0) IC17.1(A:I0) ; also sheet 1,2,4,5,7
ALU/IN/Z1/N1: IC16.8(C:I0) IC17.8(C:I0) ; also sheet 1,2,4,5,7
ALU/IN/Z1/N2: IC19.1(A:I0) IC20.1(A:I0) ; also sheet 1,2,4,5,7
ALU/IN/Z1/N3: IC19.8(C:I0) IC20.8(C:I0) ; also sheet 1,2,4,5,7
ALU/IN/Z2/N0: IC26.9(D:I) ; also sheet 1,4,5,7
ALU/IN/Z2/N1: IC26.7(C:I) ; also sheet 1,4,5,7
ALU/IN/Z2/N2: IC26.5(B:I) ; also sheet 1,4,5,7
ALU/IN/Z2/N3: IC26.3(A:I) ; also sheet 1,4,5,7
GND: C53.2 C54.2 C55.2 C56.2 C57.2 C58.2 C59.2 C60.2 C61.2 C62.2 IC16.6(B:I1) IC16.7(P:VSS) IC17.6(B:I1) IC17.7(P:VSS) IC18.7(P:VSS) IC19.7(P:VSS) IC19.11(D:O) IC20.7(P:VSS) IC21.6(B:I1) IC21.7(P:VSS) IC21.9(C:I1) IC22.6(B:I1) IC22.7(P:VSS) IC22.9(C:I1) IC23.7(P:VSS) IC24.2(A:I1) IC24.7(P:VSS) IC24.9(C:I1) IC24.11(D:O) IC25.2(A:I1) IC25.7(P:VSS) IC25.9(C:I1) IC26.14(F:I) ; also sheet 1,2,3,4,5,7,8
N$17: IC16.5(B:I0) IC17.3(A:O) IC17.5(B:I0)
N$18: IC16.3(A:O) IC18.1(A:I0)
N$30: IC16.4(B:O) IC18.2(A:I1)
N$32: IC16.13(D:I1) IC17.4(B:O) IC17.13(D:I1)
N$33: IC17.11(D:O) IC19.6(B:I1) IC20.6(B:I1)
N$38: IC16.12(D:I0) IC17.10(C:O) IC17.12(D:I0)
N$43: IC16.10(C:O) IC18.5(B:I0)
N$44: IC16.11(D:O) IC18.6(B:I1)
N$45: IC19.3(A:O) IC19.5(B:I0) IC20.5(B:I0)
N$46: IC19.4(B:O) IC19.13(D:I1) IC20.13(D:I1)
N$47: IC18.9(C:I1) IC20.4(B:O)
N$52: IC18.8(C:I0) IC20.3(A:O)
N$53: IC19.10(C:O) IC19.12(D:I0) IC20.12(D:I0)
N$57: IC18.12(D:I0) IC20.10(C:O)
N$58: IC18.13(D:I1) IC20.11(D:O)
N$59: IC21.5(B:I0) IC22.3(A:O) IC22.5(B:I0)
N$60: IC21.3(A:O) IC23.1(A:I0)
N$61: IC21.4(B:O) IC23.2(A:I1)
N$62: IC21.13(D:I1) IC22.4(B:O) IC22.13(D:I1)
N$63: IC22.11(D:O) IC24.6(B:I1) IC25.6(B:I1)
N$64: IC21.12(D:I0) IC22.10(C:O) IC22.12(D:I0)
N$65: IC21.10(C:O) IC23.5(B:I0)
N$66: IC21.11(D:O) IC23.6(B:I1)
N$67: IC24.3(A:O) IC24.5(B:I0) IC25.5(B:I0)
N$68: IC24.4(B:O) IC24.13(D:I1) IC25.13(D:I1)
N$69: IC23.9(C:I1) IC25.4(B:O)
N$70: IC23.8(C:I0) IC25.3(A:O)
N$71: IC24.10(C:O) IC24.12(D:I0) IC25.12(D:I0)
N$72: IC23.12(D:I0) IC25.10(C:O)
N$73: IC23.13(D:I1) IC25.11(D:O)
SUB/IN/Z-/N0/0: IC21.1(A:I0) IC22.1(A:I0) IC26.10(D:O)
SUB/IN/Z-/N1/0: IC21.8(C:I0) IC22.8(C:I0) IC26.6(C:O)
SUB/IN/Z-/N2/0: IC24.1(A:I0) IC25.1(A:I0) IC26.4(B:O)
SUB/IN/Z-/N3/0: IC24.8(C:I0) IC25.8(C:I0) IC26.2(A:O)
SUB/OUT/N0: IC18.3(A:O) ; also sheet 3
SUB/OUT/N1: IC18.4(B:O) ; also sheet 3
SUB/OUT/N2: IC18.10(C:O) ; also sheet 3
SUB/OUT/N3: IC18.11(D:O) ; also sheet 3
SUB/OUT/Z-/N0: IC16.2(A:I1) IC17.2(A:I1) IC23.3(A:O)
SUB/OUT/Z-/N1: IC16.9(C:I1) IC17.9(C:I1) IC23.4(B:O)
SUB/OUT/Z-/N2: IC19.2(A:I1) IC20.2(A:I1) IC23.10(C:O)
SUB/OUT/Z-/N3: IC19.9(C:I1) IC20.9(C:I1) IC23.11(D:O)
Unconnected: IC26.15(F:O)

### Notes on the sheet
- für negative zahlen weg von ground

## Sheet 7 of 8: cmpa
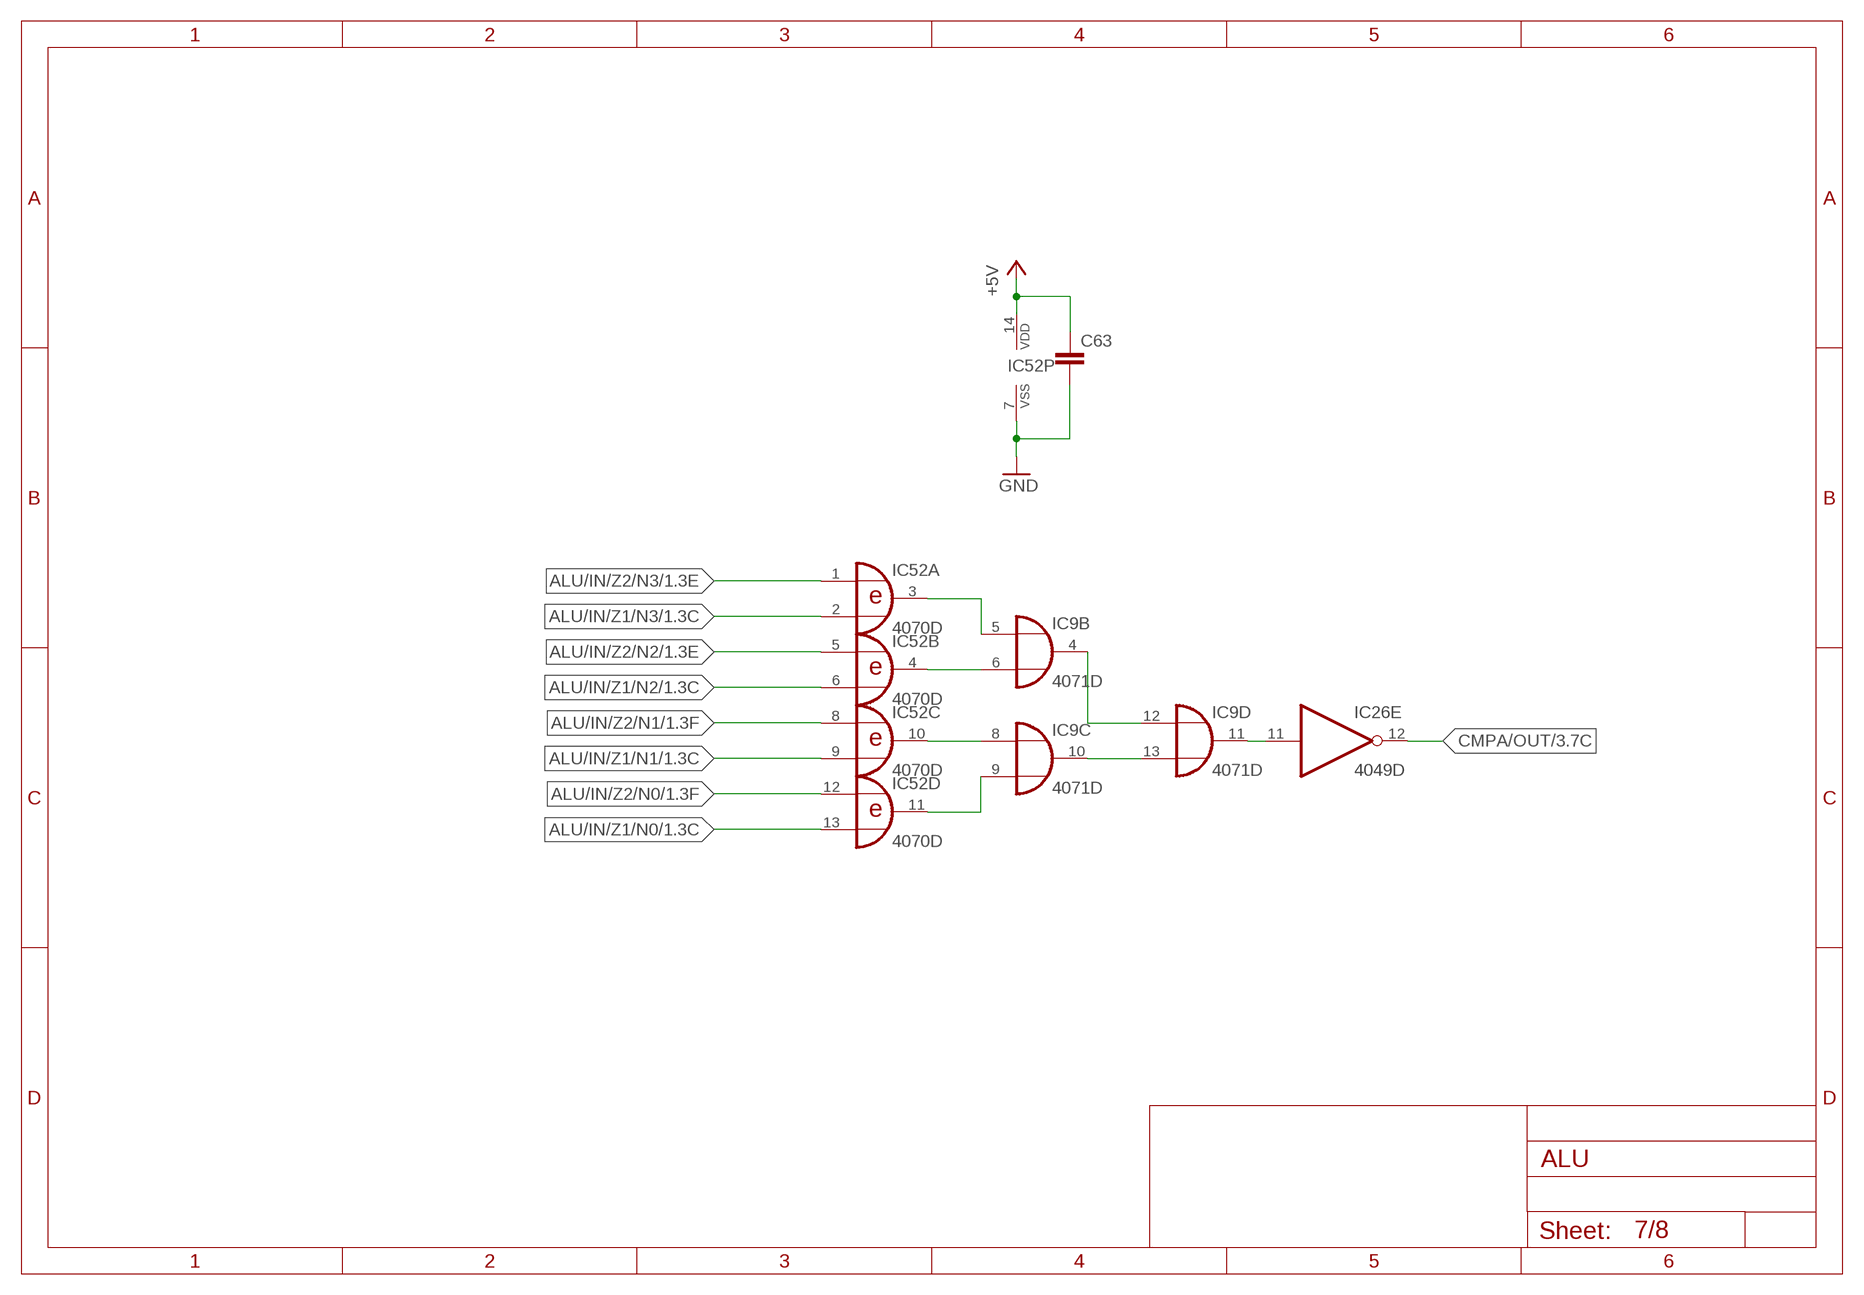
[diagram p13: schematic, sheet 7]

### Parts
C63  C-EUC0805  [C0805]
IC52  4070D  [SO14]

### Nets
+5V: C63.1 IC52.14(P:VDD) ; also sheet 1,2,3,4,5,6,8
ALU/IN/Z1/N0: IC52.13(D:I1) ; also sheet 1,2,4,5,6
ALU/IN/Z1/N1: IC52.9(C:I1) ; also sheet 1,2,4,5,6
ALU/IN/Z1/N2: IC52.6(B:I1) ; also sheet 1,2,4,5,6
ALU/IN/Z1/N3: IC52.2(A:I1) ; also sheet 1,2,4,5,6
ALU/IN/Z2/N0: IC52.12(D:I0) ; also sheet 1,4,5,6
ALU/IN/Z2/N1: IC52.8(C:I0) ; also sheet 1,4,5,6
ALU/IN/Z2/N2: IC52.5(B:I0) ; also sheet 1,4,5,6
ALU/IN/Z2/N3: IC52.1(A:I0) ; also sheet 1,4,5,6
CMPA/OUT: IC26.12(E:O) ; also sheet 3
GND: C63.2 IC52.7(P:VSS) ; also sheet 1,2,3,4,5,6,8
N$15: IC9.11(D:O) IC26.11(E:I)
N$127: IC9.9(C:I1) IC52.11(D:O)
N$128: IC9.8(C:I0) IC52.10(C:O)
N$129: IC9.6(B:I1) IC52.4(B:O)
N$130: IC9.5(B:I0) IC52.3(A:O)
N$131: IC9.10(C:O) IC9.13(D:I1)
N$132: IC9.4(B:O) IC9.12(D:I0)

## Sheet 8 of 8: Auswerter
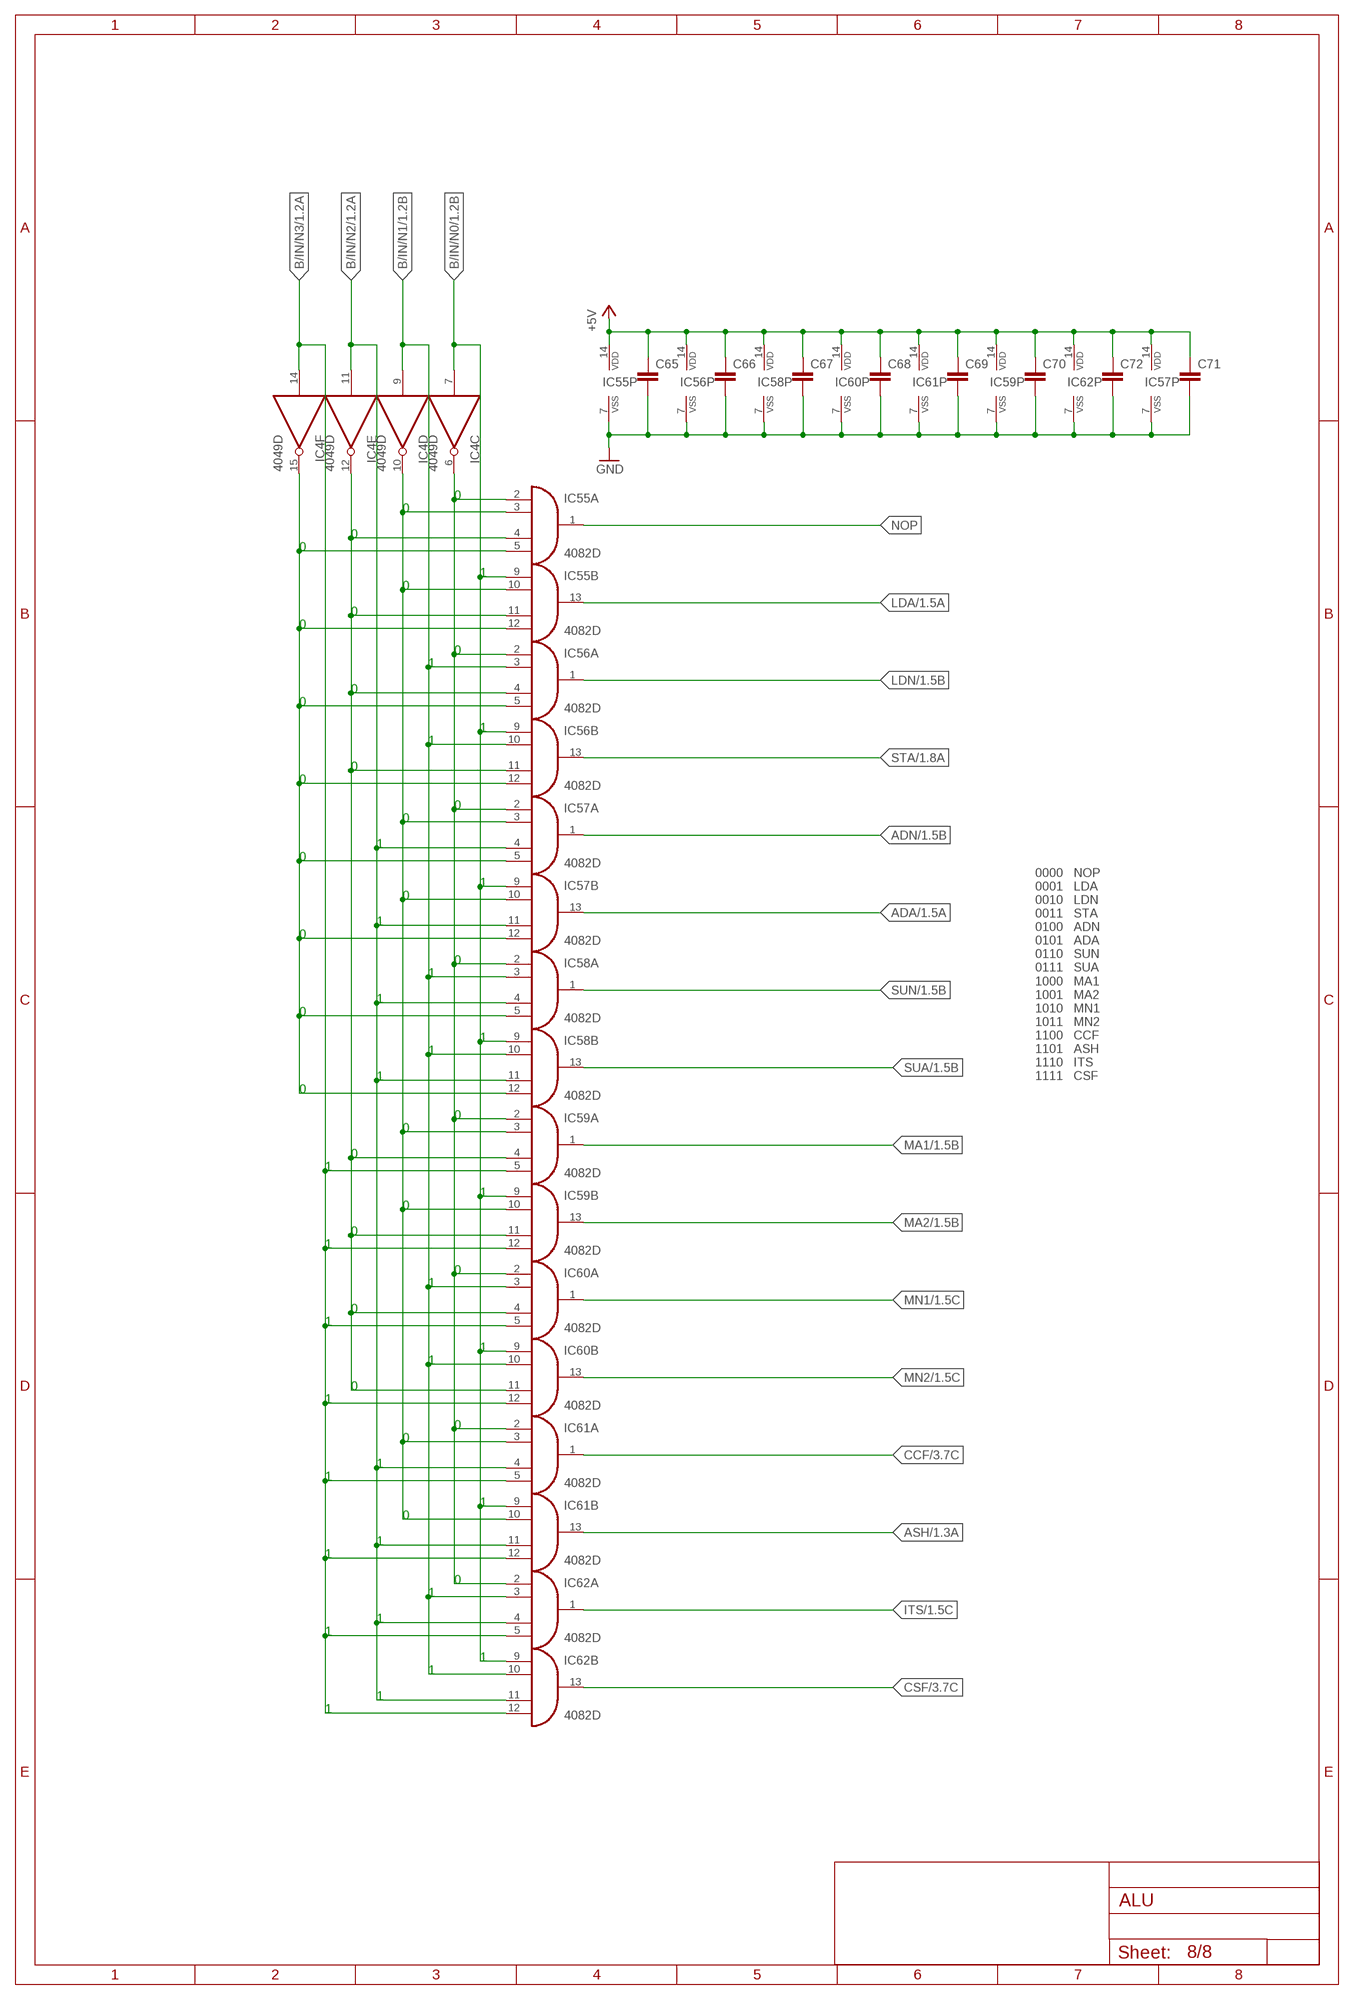
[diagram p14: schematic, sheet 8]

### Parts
C65  C-EUC0805  [C0805]
C66  C-EUC0805  [C0805]
C67  C-EUC0805  [C0805]
C68  C-EUC0805  [C0805]
C69  C-EUC0805  [C0805]
C70  C-EUC0805  [C0805]
C71  C-EUC0805  [C0805]
C72  C-EUC0805  [C0805]
IC55  4082D  [SO14]
IC56  4082D  [SO14]
IC57  4082D  [SO14]
IC58  4082D  [SO14]
IC59  4082D  [SO14]
IC60  4082D  [SO14]
IC61  4082D  [SO14]
IC62  4082D  [SO14]

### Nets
+5V: C65.1 C66.1 C67.1 C68.1 C69.1 C70.1 C71.1 C72.1 IC55.14(P:VDD) IC56.14(P:VDD) IC57.14(P:VDD) IC58.14(P:VDD) IC59.14(P:VDD) IC60.14(P:VDD) IC61.14(P:VDD) IC62.14(P:VDD) ; also sheet 1,2,3,4,5,6,7
ADA: IC57.13(B:O) ; also sheet 1
ADN: IC57.1(A:O) ; also sheet 1
ASH: IC61.13(B:O) ; also sheet 1,2
B/IN/N0: IC4.7(C:I) IC55.9(B:I0) IC56.9(B:I0) IC57.9(B:I0) IC58.9(B:I0) IC59.9(B:I0) IC60.9(B:I0) IC61.9(B:I0) IC62.9(B:I0) ; also sheet 1
B/IN/N1: IC4.9(D:I) IC56.3(A:I1) IC56.10(B:I1) IC58.3(A:I1) IC58.10(B:I1) IC60.3(A:I1) IC60.10(B:I1) IC62.3(A:I1) IC62.10(B:I1) ; also sheet 1
B/IN/N2: IC4.11(E:I) IC57.4(A:I2) IC57.11(B:I2) IC58.4(A:I2) IC58.11(B:I2) IC61.4(A:I2) IC61.11(B:I2) IC62.4(A:I2) IC62.11(B:I2) ; also sheet 1
B/IN/N3: IC4.14(F:I) IC59.5(A:I3) IC59.12(B:I3) IC60.5(A:I3) IC60.12(B:I3) IC61.5(A:I3) IC61.12(B:I3) IC62.5(A:I3) IC62.12(B:I3) ; also sheet 1
CCF: IC61.1(A:O) ; also sheet 3
CSF: IC62.13(B:O) ; also sheet 3
GND: C65.2 C66.2 C67.2 C68.2 C69.2 C70.2 C71.2 C72.2 IC55.7(P:VSS) IC56.7(P:VSS) IC57.7(P:VSS) IC58.7(P:VSS) IC59.7(P:VSS) IC60.7(P:VSS) IC61.7(P:VSS) IC62.7(P:VSS) ; also sheet 1,2,3,4,5,6,7
ITS: IC62.1(A:O) ; also sheet 1
LDA: IC55.13(B:O) ; also sheet 1
LDN: IC56.1(A:O) ; also sheet 1
MA1: IC59.1(A:O) ; also sheet 1
MA2: IC59.13(B:O) ; also sheet 1
MN1: IC60.1(A:O) ; also sheet 1
MN2: IC60.13(B:O) ; also sheet 1
N$142: IC4.6(C:O) IC55.2(A:I0) IC56.2(A:I0) IC57.2(A:I0) IC58.2(A:I0) IC59.2(A:I0) IC60.2(A:I0) IC61.2(A:I0) IC62.2(A:I0)
N$144: IC4.10(D:O) IC55.3(A:I1) IC55.10(B:I1) IC57.3(A:I1) IC57.10(B:I1) IC59.3(A:I1) IC59.10(B:I1) IC61.3(A:I1) IC61.10(B:I1)
N$146: IC4.12(E:O) IC55.4(A:I2) IC55.11(B:I2) IC56.4(A:I2) IC56.11(B:I2) IC59.4(A:I2) IC59.11(B:I2) IC60.4(A:I2) IC60.11(B:I2)
N$148: IC4.15(F:O) IC55.5(A:I3) IC55.12(B:I3) IC56.5(A:I3) IC56.12(B:I3) IC57.5(A:I3) IC57.12(B:I3) IC58.5(A:I3) IC58.12(B:I3)
NOP: IC55.1(A:O)
STA: IC56.13(B:O) ; also sheet 1
SUA: IC58.13(B:O) ; also sheet 1
SUN: IC58.1(A:O) ; also sheet 1

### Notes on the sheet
- 0
- 0
- 0
- 0
- 1
- 0
- 0
- 0
- 0
- 1
- 0
- 0
- 1
- 1
- 0
- 0
- 0
- 0
- 1
- 0
- 1
- 0
- 1
- 0
- 0
- 1
- 1
- 0
- 1
- 1
- 1
- 0000   NOP
  0001   LDA
  0010   LDN
  0011   STA
  0100   ADN
  0101   ADA
  0110   SUN
  0111   SUA
  1000   MA1
  1001   MA2
  1010   MN1
  1011   MN2
  1100   CCF
  1101   ASH
  1110   ITS
  1111   CSF
- 0
- 0
- 0
- 0
- 1
- 1
- 0
- 0
- 1
- 0
- 1
- 0
- 1
- 1
- 1
- 0
- 1
- 0
- 0
- 1
- 1
- 1
- 0
- 1
- 1
- 0
- 1
- 1
- 1
- 1
- 1
- 1
- 1

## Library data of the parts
+5V CARRY CHECK CLK GND R RCLK SAME W = pinhead:PINHD-1X1: PIN HEADER
ADRESS BEFEHL IN/NUMBER NUMBER REGISTER/OUT = pinhead:PINHD-1X4: PIN HEADER
C1-C24 C26 C27 C29-C63 C65-C72 = rcl:C-EU: CAPACITOR, European symbol; SPICEPREFIX: C
IC1 IC3 IC5 IC7 IC47 = 40xx:4027: Dual JK FLIP FLOP
IC2 IC4 IC26 = 40xx:4049: Hex inverting BUFFER
IC6 IC10 IC12 IC15 IC16 IC20 IC21 IC25 IC27-IC31 IC35 IC36 IC40 IC41 IC45 IC48-IC51 IC63-IC65 = 40xx:4081: Quad 2-input AND
IC8 IC9 IC13 IC18 IC23 IC33 IC38 IC43 IC67-IC70 = 40xx:4071: Quad 2-input OR
IC11 IC14 IC17 IC19 IC22 IC24 IC32 IC34 IC37 IC39 IC42 IC44 IC52 = 40xx:4070: Quad 2-input XOR
IC53 IC54 IC66 = 40xx:4072: Dual 4-input OR
IC55-IC62 = 40xx:4082: Dual 4-input AND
